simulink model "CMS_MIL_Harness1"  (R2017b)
settings: Solver=FixedStepDiscrete  StartTime=0.0  StopTime=23  FixedStep=0.01  RelTol=1e-3  EnableMultiTasking=on
undefined symbols (not defined in the file): sigbuilder_block
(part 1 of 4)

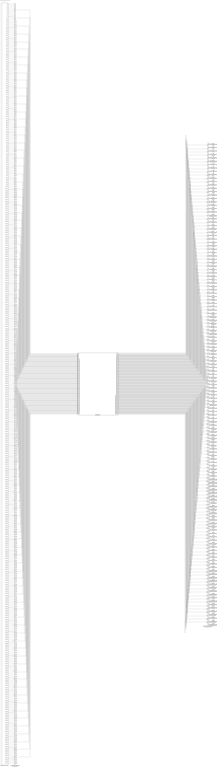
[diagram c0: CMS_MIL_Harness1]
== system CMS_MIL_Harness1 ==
  CMS_MIL : ModelReference  ModelNameDialog=CMS_MIL  SimulationMode=Normal  ModelReferenceVersion='M109C106'
  Harness Inputs : Subsystem  Tag=STV Subsys  LoadFcn=sigbuilder_block('load');  StartFcn=sigbuilder_block('start');  StopFcn=sigbuilder_block('stop');  ClipboardFcn=sigbuilder_block('clipboard');  mask(Sigbuilder block){tuvar=[0:10]}
      mask init:
      | if ~strcmp(get_param(bdroot(gcb),'SimulationStatus'),'stopped'),tuvar = sigbuilder_block('maskInit'); end
  Input Conversion Subsystem : Subsystem  Tag=__SLT_ICS__  Description=Signal spec. and routing
  Output Conversion Subsystem : Subsystem  Tag=__SLT_OCS__  Description=Signal spec. and routing
  GeCMS_HVConnSt_enum : Outport  OutDataTypeStr=uint8  PortDimensions=[1]
  GbCMS_NegCtlSt_flg : Outport  Port=2  OutDataTypeStr=boolean  PortDimensions=[1]
  GbCMS_PosCtlSt_flg : Outport  Port=3  OutDataTypeStr=boolean  PortDimensions=[1]
  GbCMS_ChrgPosCtlSt_flg : Outport  Port=4  OutDataTypeStr=boolean  PortDimensions=[1]
  GbCMS_ChrgNegCtlSt_flg : Outport  Port=5  OutDataTypeStr=boolean  PortDimensions=[1]
  GeCMS_RelStuckClosed_enum : Outport  Port=6  OutDataTypeStr=uint8  PortDimensions=[1]
  GcCMS_PackVolt_V : Outport  Port=7  OutDataTypeStr=fixdt('ufix16_Sp1')  PortDimensions=[1]
  GbCMS_PreChrgCtlSt_flg : Outport  Port=8  OutDataTypeStr=boolean  PortDimensions=[1]
  GcCMS_BattCurr_A : Outport  Port=9  OutDataTypeStr=fixdt('ufix16_Sp1_Bn700')  PortDimensions=[1]
  GbCMS_Kl15WkUp_flg : Outport  Port=10  OutDataTypeStr=boolean  PortDimensions=[1]
  GbCMS_ThmRunAway_flg : Outport  Port=11  OutDataTypeStr=boolean  PortDimensions=[1]
  GcCMS_CoolTempIn_C : Outport  Port=12  OutDataTypeStr=fixdt('ufix8_Bn40')  PortDimensions=[1]
  GcCMS_CoolTempOut_C : Outport  Port=13  OutDataTypeStr=fixdt('ufix8_Bn40')  PortDimensions=[1]
  GcCMS_CoolPwrReq_W : Outport  Port=14  OutDataTypeStr=fixdt('ufix16_Sp1')  PortDimensions=[1]
  GcCMS_HeatPwrReq_W : Outport  Port=15  OutDataTypeStr=fixdt('ufix16_Sp1')  PortDimensions=[1]
  GeCMS_CoolReq_enum : Outport  Port=16  OutDataTypeStr=uint8  PortDimensions=[1]
  GeCMS_HeatReq_enum : Outport  Port=17  OutDataTypeStr=uint8  PortDimensions=[1]
  GcCMS_PeakCurrDisCh_A : Outport  Port=18  OutDataTypeStr=fixdt('ufix16_Sp1')  PortDimensions=[1]
  GcCMS_PeakCurrCh_A : Outport  Port=19  OutDataTypeStr=fixdt('ufix16_Sp1_Bn1500')  PortDimensions=[1]
  GcCMS_PeakVoltDisCh_V : Outport  Port=20  OutDataTypeStr=uint16  PortDimensions=[1]
  GcCMS_PeakVoltCh_V : Outport  Port=21  OutDataTypeStr=uint16  PortDimensions=[1]
  GeCMS_Thm_propagat_enum : Outport  Port=22  OutDataTypeStr=uint8  PortDimensions=[1]
  GcCMS_ClntTgtTemp_C : Outport  Port=23  OutDataTypeStr=fixdt('ufix8_Bn40')  PortDimensions=[1]
  GcCMS_HtTgtTemp_C : Outport  Port=24  OutDataTypeStr=fixdt('ufix8_Bn40')  PortDimensions=[1]
  GcCMS_MaxCellVolt_V : Outport  Port=25  OutDataTypeStr=fixdt('ufix16_Sp001')  PortDimensions=[1]
  GcCMS_BusbarTempMax_C : Outport  Port=26  OutDataTypeStr=fixdt('ufix8_Bn40')  PortDimensions=[1]
  GcCMS_BusbarTempMin_C : Outport  Port=27  OutDataTypeStr=fixdt('ufix8_Bn40')  PortDimensions=[1]
  GcCMS_MinCellVolt_V : Outport  Port=28  OutDataTypeStr=fixdt('ufix16_Sp001')  PortDimensions=[1]
  GbCMS_ChrgCmd_flg : Outport  Port=29  OutDataTypeStr=boolean  PortDimensions=[1]
  GcCMS_ActPwrChrg_Kw : Outport  Port=30  OutDataTypeStr=fixdt('ufix16_Sp1')  PortDimensions=[1]
  GcCMS_MaxVoltChrg_V : Outport  Port=31  OutDataTypeStr=fixdt('ufix16_Sp1')  PortDimensions=[1]
  GcCMS_ReqVoltChrg_V : Outport  Port=32  OutDataTypeStr=fixdt('ufix16_Sp1')  PortDimensions=[1]
  GcCMS_ReqCurrChrg_A : Outport  Port=33  OutDataTypeStr=fixdt('ufix16_Sp1_Bn700')  PortDimensions=[1]
  GbCMS_ObcRdyReq_flg : Outport  Port=34  OutDataTypeStr=boolean  PortDimensions=[1]
  GbCMS_DischgCmd_flg : Outport  Port=35  OutDataTypeStr=boolean  PortDimensions=[1]
  GeCMS_BmsSt_enum : Outport  Port=36  OutDataTypeStr=uint8  PortDimensions=[1]
  GeCMS_BmsSelfChk_enum : Outport  Port=37  OutDataTypeStr=uint8  PortDimensions=[1]
  GeCMS_IsoFault_enum : Outport  Port=38  OutDataTypeStr=uint8  PortDimensions=[1]
  GcCMS_SocDspl_pct : Outport  Port=39  OutDataTypeStr=uint8  PortDimensions=[1]
  GbCMS_HvilOpenFault_flg : Outport  Port=40  OutDataTypeStr=boolean  PortDimensions=[1]
  GeCMS_FltLvl_enum : Outport  Port=41  OutDataTypeStr=uint8  PortDimensions=[1]
  GeCMS_V2xMod_enum : Outport  Port=42  OutDataTypeStr=uint8  PortDimensions=[1]
  GcCMS_ChgSOCset_pct : Outport  Port=43  OutDataTypeStr=fixdt('ufix8_B80')  PortDimensions=[1]
  GcCMS_BattSoh_pct : Outport  Port=44  OutDataTypeStr=uint8  PortDimensions=[1]
  GcCMS_SOCA_pct : Outport  Port=45  OutDataTypeStr=uint8  PortDimensions=[1]
  GeCMS_IviDischg_enum : Outport  Port=46  OutDataTypeStr=uint8  PortDimensions=[1]
  GcCMS_PackCurLem_A : Outport  Port=47  OutDataTypeStr=fixdt('ufix16_Bn1023')  PortDimensions=[1]
  GcCMS_BattInVolt_V : Outport  Port=48  OutDataTypeStr=fixdt('ufix16_Sp1')  PortDimensions=[1]
  GbCMS_BalSt_flg : Outport  Port=49  OutDataTypeStr=boolean  PortDimensions=[1]
  GbCMS_BalVlg_flg : Outport  Port=50  OutDataTypeStr=boolean  PortDimensions=[1]
  GbCMS_VcuPwrUpReq_flg : Outport  Port=51  OutDataTypeStr=boolean  PortDimensions=[1]
  GbCMS_VcuPwrUpReqVld_flg : Outport  Port=52  OutDataTypeStr=boolean  PortDimensions=[1]
  GcCMS_ConstCurrDisChMax_A : Outport  Port=53  OutDataTypeStr=fixdt('ufix16_Sp1')  PortDimensions=[1]
  GcCMS_ConstCurrChMax_A : Outport  Port=54  OutDataTypeStr=fixdt('ufix16_Sp1_Bn700')  PortDimensions=[1]
  GbCMS_PwrDownReq_flg : Outport  Port=55  OutDataTypeStr=boolean  PortDimensions=[1]
  GbCMS_PwrDownReqVld_flg : Outport  Port=56  OutDataTypeStr=boolean  PortDimensions=[1]
  GeCMS_ChrgPreThmMode_enum : Outport  Port=57  OutDataTypeStr=uint8  PortDimensions=[1]
  GeCMS_ElockReq_enum : Outport  Port=58  OutDataTypeStr=uint8  PortDimensions=[1]
  GeCMS_PreThmReq_enum : Outport  Port=59  OutDataTypeStr=uint8  PortDimensions=[1]
  GcCMS_PeakPwrDisCh_Kw : Outport  Port=60  OutDataTypeStr=fixdt('ufix16_Sp1')  PortDimensions=[1]
  GcCMS_PeakPwrCh_Kw : Outport  Port=61  OutDataTypeStr=fixdt('ufix16_Sp1')  PortDimensions=[1]
  GcCMS_ConstPwrDisCh_Kw : Outport  Port=62  OutDataTypeStr=fixdt('ufix16_Sp1')  PortDimensions=[1]
  GcCMS_ConstPwrCh_Kw : Outport  Port=63  OutDataTypeStr=fixdt('ufix16_Sp1')  PortDimensions=[1]
  GcCMS_ResIso_Kohm : Outport  Port=64  OutDataTypeStr=uint16  PortDimensions=[1]
  GcCMS_ChrgRemTime_Min : Outport  Port=65  OutDataTypeStr=uint16  PortDimensions=[1]
  GeCMS_ACPlugCnnt_enum : Outport  Port=66  OutDataTypeStr=uint8  PortDimensions=[1]
  GbCMS_BattFull_flg : Outport  Port=67  OutDataTypeStr=boolean  PortDimensions=[1]
  GbCMS_WarnLamp_flg : Outport  Port=68  OutDataTypeStr=boolean  PortDimensions=[1]
  GbCMS_SerLamp_flg : Outport  Port=69  OutDataTypeStr=boolean  PortDimensions=[1]
  GbCMS_TempDiffWarn_flg : Outport  Port=70  OutDataTypeStr=boolean  PortDimensions=[1]
  GbCMS_OverChrgWarn_flg : Outport  Port=71  OutDataTypeStr=boolean  PortDimensions=[1]
  GbCMS_ConsisWarn_flg : Outport  Port=72  OutDataTypeStr=boolean  PortDimensions=[1]
  GbCMS_MishWarn_flg : Outport  Port=73  OutDataTypeStr=boolean  PortDimensions=[1]
  GbCMS_SocHopWarn_flg : Outport  Port=74  OutDataTypeStr=boolean  PortDimensions=[1]
  GbCMS_SocHighWarn_flg : Outport  Port=75  OutDataTypeStr=boolean  PortDimensions=[1]
  GbCMS_SocLowWarn_flg : Outport  Port=76  OutDataTypeStr=boolean  PortDimensions=[1]
  GbCMS_OTAModeSt_flg : Outport  Port=77  OutDataTypeStr=boolean  PortDimensions=[1]
  GeCMS_AcDcConnBoth_enum : Outport  Port=78  OutDataTypeStr=uint8  PortDimensions=[1]
  GbCMS_CellUvFlt_flg : Outport  Port=79  OutDataTypeStr=boolean  PortDimensions=[1]
  GbCMS_CellOvFlt_flg : Outport  Port=80  OutDataTypeStr=boolean  PortDimensions=[1]
  GbCMS_PackUvFlt_flg : Outport  Port=81  OutDataTypeStr=boolean  PortDimensions=[1]
  GbCMS_PackOvFlt_flg : Outport  Port=82  OutDataTypeStr=boolean  PortDimensions=[1]
  GbCMS_TempHighWarn_flg : Outport  Port=83  OutDataTypeStr=boolean  PortDimensions=[1]
  GcCMS_RealSoc_pct : Outport  Port=84  OutDataTypeStr=uint8  PortDimensions=[1]
  GeCMS_DCPlugConn_enum : Outport  Port=85  OutDataTypeStr=uint8  PortDimensions=[1]
  GeCMS_ACChgMode_enum : Outport  Port=86  OutDataTypeStr=uint8  PortDimensions=[1]
  GeCMS_DCChgMode_enum : Outport  Port=87  OutDataTypeStr=uint8  PortDimensions=[1]
  GcCMS_BattTempAvrg_C : Outport  Port=88  OutDataTypeStr=fixdt('ufix8_Bn40')  PortDimensions=[1]
  GcCMS_BattNrmEnrg_kwh : Outport  Port=89  OutDataTypeStr=fixdt('ufix16_Sp01')  PortDimensions=[1]
  GbCMS_BattTempFault_flg : Outport  Port=90  OutDataTypeStr=boolean  PortDimensions=[1]
  GcCMS_BattSoe_kwh : Outport  Port=91  OutDataTypeStr=fixdt('ufix16_Sp1')  PortDimensions=[1]
  GbCMS_IsoChkSt_flg : Outport  Port=92  OutDataTypeStr=boolean  PortDimensions=[1]
  GcCMS_BattTempMax_C : Outport  Port=93  OutDataTypeStr=fixdt('ufix8_Bn40')  PortDimensions=[1]
  GcCMS_BattTempMin_C : Outport  Port=94  OutDataTypeStr=fixdt('ufix8_Bn40')  PortDimensions=[1]
  GcCMS_FuseVolt_V : Outport  Port=95  OutDataTypeStr=fixdt('ufix8_E1')  PortDimensions=[1]
  GcCMS_ChrgAccum_Ah : Outport  Port=96  OutDataTypeStr=uint8  PortDimensions=[1]
  GbCMS_DChgStVoltOut_flg : Outport  Port=97  OutDataTypeStr=boolean  PortDimensions=[1]
  GcCMS_DChrgVoltReq_V : Outport  Port=98  OutDataTypeStr=fixdt('ufix16_Sp1')  PortDimensions=[1]
  GcCMS_DChrgCurrReq_A : Outport  Port=99  OutDataTypeStr=fixdt('ufix16_Sp1_Bn400')  PortDimensions=[1]
  GcCMS_DChrgRchSocLmt_numb : Outport  Port=100  OutDataTypeStr=uint8  PortDimensions=[1]
  GcCMS_DChrgRchPackVoltLmt_numb : Outport  Port=101  OutDataTypeStr=uint8  PortDimensions=[1]
  GcCMS_DChrgRchCellVoltLmt_numb : Outport  Port=102  OutDataTypeStr=uint8  PortDimensions=[1]
  GcCMS_DChrgChrgerActStop_numb : Outport  Port=103  OutDataTypeStr=uint8  PortDimensions=[1]
  GcCMS_DChrgBattInsulationErr_numb : Outport  Port=104  OutDataTypeStr=uint8  PortDimensions=[1]
  GcCMS_DChrgOutpCnntOvrTempErr_numb : Outport  Port=105  OutDataTypeStr=uint8  PortDimensions=[1]
  GcCMS_PcbOvrTempErr_numb : Outport  Port=106  OutDataTypeStr=uint8  PortDimensions=[1]
  GcCMS_ChrgCnntErr_numb : Outport  Port=107  OutDataTypeStr=uint8  PortDimensions=[1]
  GcCMS_BattOvrTempErr_numb : Outport  Port=108  OutDataTypeStr=uint8  PortDimensions=[1]
  GcCMS_MainRelayErr_numb : Outport  Port=109  OutDataTypeStr=uint8  PortDimensions=[1]
  GcCMS_CC2ChkVoltErr_numb : Outport  Port=110  OutDataTypeStr=uint8  PortDimensions=[1]
  GcCMS_OtherErr_numb : Outport  Port=111  OutDataTypeStr=uint8  PortDimensions=[1]
  GcCMS_ChrgCurrAbnrm_numb : Outport  Port=112  OutDataTypeStr=uint8  PortDimensions=[1]
  GcCMS_ChrgVoltAbnrm_numb : Outport  Port=113  OutDataTypeStr=uint8  PortDimensions=[1]
  GcCMS_CellVoltCnt_numb : Outport  Port=114  OutDataTypeStr=uint8  PortDimensions=[1]
  GcCMS_CellVolt1_V : Outport  Port=115  OutDataTypeStr=fixdt('ufix16_Sp001')  PortDimensions=[1]
  GcCMS_CellVolt2_V : Outport  Port=116  OutDataTypeStr=fixdt('ufix16_Sp001')  PortDimensions=[1]
  GcCMS_CellVolt3_V : Outport  Port=117  OutDataTypeStr=fixdt('ufix16_Sp001')  PortDimensions=[1]
  GcCMS_CellVolt4_V : Outport  Port=118  OutDataTypeStr=fixdt('ufix16_Sp001')  PortDimensions=[1]
  GcCMS_CellTempCnt_numb : Outport  Port=119  OutDataTypeStr=uint8  PortDimensions=[1]
  GcCMS_CellTemp1_C : Outport  Port=120  OutDataTypeStr=fixdt('ufix8_Bn40')  PortDimensions=[1]
  GcCMS_CellTemp2_C : Outport  Port=121  OutDataTypeStr=fixdt('ufix8_Bn40')  PortDimensions=[1]
  GcCMS_CellTemp3_C : Outport  Port=122  OutDataTypeStr=fixdt('ufix8_Bn40')  PortDimensions=[1]
  GcCMS_CellTemp4_C : Outport  Port=123  OutDataTypeStr=fixdt('ufix8_Bn40')  PortDimensions=[1]
  GcCMS_CellTemp5_C : Outport  Port=124  OutDataTypeStr=fixdt('ufix8_Bn40')  PortDimensions=[1]
  GcCMS_CellTemp6_C : Outport  Port=125  OutDataTypeStr=fixdt('ufix8_Bn40')  PortDimensions=[1]
  GcCMS_CellTemp7_C : Outport  Port=126  OutDataTypeStr=fixdt('ufix8_Bn40')  PortDimensions=[1]
  GcCMS_MaxCellVoltNumb_numb : Outport  Port=127  OutDataTypeStr=uint8  PortDimensions=[1]
  GcCMS_MinCellVoltNumb_numb : Outport  Port=128  OutDataTypeStr=uint8  PortDimensions=[1]
  GcCMS_MaxCellTempNumb_numb : Outport  Port=129  OutDataTypeStr=uint8  PortDimensions=[1]
  GcCMS_MinCellTempNumb_numb : Outport  Port=130  OutDataTypeStr=uint8  PortDimensions=[1]
  GcCMS_MaxVoltNumb_numb : Outport  Port=131  OutDataTypeStr=uint8  PortDimensions=[1]
  GcCMS_MinVoltNumb_numb : Outport  Port=132  OutDataTypeStr=uint8  PortDimensions=[1]
  GcCMS_MaxTempNumb_numb : Outport  Port=133  OutDataTypeStr=uint8  PortDimensions=[1]
  GcCMS_MinTempNumb_numb : Outport  Port=134  OutDataTypeStr=uint8  PortDimensions=[1]
  GeCMS_ChgMode_enum : Outport  Port=135  OutDataTypeStr=uint8  PortDimensions=[1]
  GeCMS_DChrgModeDebug_enum : Outport  Port=136  OutDataTypeStr=uint8  PortDimensions=[1]
  GbCMS_DChrgWkUp_flg : Outport  Port=137  OutDataTypeStr=boolean  PortDimensions=[1]
  GeCMS_EvccMode_enum : Outport  Port=138  OutDataTypeStr=uint8  PortDimensions=[1]
  GeCMS_AChrgObsr_enum : Outport  Port=139  OutDataTypeStr=uint8  PortDimensions=[1]
  GeCMS_PreThmObsvr_enum : Outport  Port=140  OutDataTypeStr=uint8  PortDimensions=[1]
  GbCMS_StartCanSend_flg : Outport  Port=141  OutDataTypeStr=boolean  PortDimensions=[1]
  GeCMS_AppChgMode_enum : Outport  Port=142  OutDataTypeStr=uint8  PortDimensions=[1]
  GeCMS_DCchgIsolationFault_enum : Outport  Port=143  OutDataTypeStr=uint8  PortDimensions=[1]
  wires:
  Harness Inputs/1(GeCTC_CtrCtlState_enum) -> Input Conversion Subsystem/1(Inport_1)
  Harness Inputs/2(GbCTC_NegCtlState_flg) -> Input Conversion Subsystem/2(Inport_2)
  Harness Inputs/3(GbCTC_PosCtlState_flg) -> Input Conversion Subsystem/3(Inport_3)
  Harness Inputs/4(GbCTC_DCPosChrgCtlState_flg) -> Input Conversion Subsystem/4(Inport_4)
  Harness Inputs/5(GbCTC_DCNegChrgCtlState_flg) -> Input Conversion Subsystem/5(Inport_5)
  Harness Inputs/6(GcHDP_PackVolt_V) -> Input Conversion Subsystem/6(Inport_6)
  Harness Inputs/7(GbCTC_PreChrgCtlState_flg) -> Input Conversion Subsystem/7(Inport_7)
  Harness Inputs/8(GcHDP_PackCrnt_A) -> Input Conversion Subsystem/8(Inport_8)
  Harness Inputs/9(GbWSM_Kl15WkUpPrs_flg) -> Input Conversion Subsystem/9(Inport_9)
  Harness Inputs/10(GcCDP_MinCellVolt_mV) -> Input Conversion Subsystem/10(Inport_10)
  Harness Inputs/11(GcCDP_MaxCellVolt_mV) -> Input Conversion Subsystem/11(Inport_11)
  Harness Inputs/12(GbACC_ObcChrgCmd_flg) -> Input Conversion Subsystem/12(Inport_12)
  Harness Inputs/13(GcACC_ACChrgVoltRqst_V) -> Input Conversion Subsystem/13(Inport_13)
  Harness Inputs/14(GcACC_ACChrgCrntRqst_A) -> Input Conversion Subsystem/14(Inport_14)
  Harness Inputs/15(GbACC_ACChrgRqst_flg) -> Input Conversion Subsystem/15(Inport_15)
  Harness Inputs/16(GeCTC_CtrCtlConnMode_enum) -> Input Conversion Subsystem/16(Inport_16)
  Harness Inputs/17(GbMSM_SelfCheck_flg) -> Input Conversion Subsystem/17(Inport_17)
  Harness Inputs/18(GcSOC_DispSOC_pct) -> Input Conversion Subsystem/18(Inport_18)
  Harness Inputs/19(GbISP_TFHvilLFlt_flg) -> Input Conversion Subsystem/19(Inport_19)
  Harness Inputs/20(GeFTC_FltLvlOnCAN_enum) -> Input Conversion Subsystem/20(Inport_20)
  Harness Inputs/21(GcSOH_PackSOH_pct) -> Input Conversion Subsystem/21(Inport_21)
  Harness Inputs/22(GcSOC_PackSOC_pct) -> Input Conversion Subsystem/22(Inport_22)
  Harness Inputs/23(GcHDP_HallCrnt_A) -> Input Conversion Subsystem/23(Inport_23)
  Harness Inputs/24(GbMSM_SelfChckMaxTiReach_flg) -> Input Conversion Subsystem/24(Inport_24)
  Harness Inputs/25(GaCBC_CellBalCtlCmd_flg(1)) -> Input Conversion Subsystem/25(Inport_25)
  Harness Inputs/26(GaCBC_CellBalCtlCmd_flg(2)) -> Input Conversion Subsystem/26(Inport_26)
  Harness Inputs/27(GaCBC_CellBalCtlCmd_flg(3)) -> Input Conversion Subsystem/27(Inport_27)
  Harness Inputs/28(GaCBC_CellBalCtlCmd_flg(4)) -> Input Conversion Subsystem/28(Inport_28)
  Harness Inputs/29(GaCBC_CellBalCtlCmd_flg(5)) -> Input Conversion Subsystem/29(Inport_29)
  Harness Inputs/30(GaCBC_CellBalCtlCmd_flg(6)) -> Input Conversion Subsystem/30(Inport_30)
  Harness Inputs/31(GaCBC_CellBalCtlCmd_flg(7)) -> Input Conversion Subsystem/31(Inport_31)
  Harness Inputs/32(GaCBC_CellBalCtlCmd_flg(8)) -> Input Conversion Subsystem/32(Inport_32)
  Harness Inputs/33(GaCBC_CellBalCtlCmd_flg(9)) -> Input Conversion Subsystem/33(Inport_33)
  Harness Inputs/34(GaCBC_CellBalCtlCmd_flg(10)) -> Input Conversion Subsystem/34(Inport_34)
  Harness Inputs/35(GaCBC_CellBalCtlCmd_flg(11)) -> Input Conversion Subsystem/35(Inport_35)
  Harness Inputs/36(GaCBC_CellBalCtlCmd_flg(12)) -> Input Conversion Subsystem/36(Inport_36)
  Harness Inputs/37(GaCBC_CellBalCtlCmd_flg(13)) -> Input Conversion Subsystem/37(Inport_37)
  Harness Inputs/38(GaCBC_CellBalCtlCmd_flg(14)) -> Input Conversion Subsystem/38(Inport_38)
  Harness Inputs/39(GaCBC_CellBalCtlCmd_flg(15)) -> Input Conversion Subsystem/39(Inport_39)
  Harness Inputs/40(GaCBC_CellBalCtlCmd_flg(16)) -> Input Conversion Subsystem/40(Inport_40)
  Harness Inputs/41(GaCBC_CellBalCtlCmd_flg(17)) -> Input Conversion Subsystem/41(Inport_41)
  Harness Inputs/42(GaCBC_CellBalCtlCmd_flg(18)) -> Input Conversion Subsystem/42(Inport_42)
  Harness Inputs/43(GaCBC_CellBalCtlCmd_flg(19)) -> Input Conversion Subsystem/43(Inport_43)
  Harness Inputs/44(GaCBC_CellBalCtlCmd_flg(20)) -> Input Conversion Subsystem/44(Inport_44)
  Harness Inputs/45(GaCBC_CellBalCtlCmd_flg(21)) -> Input Conversion Subsystem/45(Inport_45)
  Harness Inputs/46(GaCBC_CellBalCtlCmd_flg(22)) -> Input Conversion Subsystem/46(Inport_46)
  Harness Inputs/47(GaCBC_CellBalCtlCmd_flg(23)) -> Input Conversion Subsystem/47(Inport_47)
  Harness Inputs/48(GaCBC_CellBalCtlCmd_flg(24)) -> Input Conversion Subsystem/48(Inport_48)
  Harness Inputs/49(GaCBC_CellBalCtlCmd_flg(25)) -> Input Conversion Subsystem/49(Inport_49)
  Harness Inputs/50(GaCBC_CellBalCtlCmd_flg(26)) -> Input Conversion Subsystem/50(Inport_50)
  Harness Inputs/51(GaCBC_CellBalCtlCmd_flg(27)) -> Input Conversion Subsystem/51(Inport_51)
  Harness Inputs/52(GaCBC_CellBalCtlCmd_flg(28)) -> Input Conversion Subsystem/52(Inport_52)
  Harness Inputs/53(GaCBC_CellBalCtlCmd_flg(29)) -> Input Conversion Subsystem/53(Inport_53)
  Harness Inputs/54(GaCBC_CellBalCtlCmd_flg(30)) -> Input Conversion Subsystem/54(Inport_54)
  Harness Inputs/55(GaCBC_CellBalCtlCmd_flg(31)) -> Input Conversion Subsystem/55(Inport_55)
  Harness Inputs/56(GaCBC_CellBalCtlCmd_flg(32)) -> Input Conversion Subsystem/56(Inport_56)
  Harness Inputs/57(GaCBC_CellBalCtlCmd_flg(33)) -> Input Conversion Subsystem/57(Inport_57)
  Harness Inputs/58(GaCBC_CellBalCtlCmd_flg(34)) -> Input Conversion Subsystem/58(Inport_58)
  Harness Inputs/59(GaCBC_CellBalCtlCmd_flg(35)) -> Input Conversion Subsystem/59(Inport_59)
  Harness Inputs/60(GaCBC_CellBalCtlCmd_flg(36)) -> Input Conversion Subsystem/60(Inport_60)
  Harness Inputs/61(GaCBC_CellBalCtlCmd_flg(37)) -> Input Conversion Subsystem/61(Inport_61)
  Harness Inputs/62(GaCBC_CellBalCtlCmd_flg(38)) -> Input Conversion Subsystem/62(Inport_62)
  Harness Inputs/63(GaCBC_CellBalCtlCmd_flg(39)) -> Input Conversion Subsystem/63(Inport_63)
  Harness Inputs/64(GaCBC_CellBalCtlCmd_flg(40)) -> Input Conversion Subsystem/64(Inport_64)
  Harness Inputs/65(GaCBC_CellBalCtlCmd_flg(41)) -> Input Conversion Subsystem/65(Inport_65)
  Harness Inputs/66(GaCBC_CellBalCtlCmd_flg(42)) -> Input Conversion Subsystem/66(Inport_66)
  Harness Inputs/67(GaCBC_CellBalCtlCmd_flg(43)) -> Input Conversion Subsystem/67(Inport_67)
  Harness Inputs/68(GaCBC_CellBalCtlCmd_flg(44)) -> Input Conversion Subsystem/68(Inport_68)
  Harness Inputs/69(GaCBC_CellBalCtlCmd_flg(45)) -> Input Conversion Subsystem/69(Inport_69)
  Harness Inputs/70(GaCBC_CellBalCtlCmd_flg(46)) -> Input Conversion Subsystem/70(Inport_70)
  Harness Inputs/71(GaCBC_CellBalCtlCmd_flg(47)) -> Input Conversion Subsystem/71(Inport_71)
  Harness Inputs/72(GaCBC_CellBalCtlCmd_flg(48)) -> Input Conversion Subsystem/72(Inport_72)
  Harness Inputs/73(GaCBC_CellBalCtlCmd_flg(49)) -> Input Conversion Subsystem/73(Inport_73)
  Harness Inputs/74(GaCBC_CellBalCtlCmd_flg(50)) -> Input Conversion Subsystem/74(Inport_74)
  Harness Inputs/75(GaCBC_CellBalCtlCmd_flg(51)) -> Input Conversion Subsystem/75(Inport_75)
  Harness Inputs/76(GaCBC_CellBalCtlCmd_flg(52)) -> Input Conversion Subsystem/76(Inport_76)
  Harness Inputs/77(GaCBC_CellBalCtlCmd_flg(53)) -> Input Conversion Subsystem/77(Inport_77)
  Harness Inputs/78(GaCBC_CellBalCtlCmd_flg(54)) -> Input Conversion Subsystem/78(Inport_78)
  Harness Inputs/79(GaCBC_CellBalCtlCmd_flg(55)) -> Input Conversion Subsystem/79(Inport_79)
  Harness Inputs/80(GaCBC_CellBalCtlCmd_flg(56)) -> Input Conversion Subsystem/80(Inport_80)
  Harness Inputs/81(GaCBC_CellBalCtlCmd_flg(57)) -> Input Conversion Subsystem/81(Inport_81)
  Harness Inputs/82(GaCBC_CellBalCtlCmd_flg(58)) -> Input Conversion Subsystem/82(Inport_82)
  Harness Inputs/83(GaCBC_CellBalCtlCmd_flg(59)) -> Input Conversion Subsystem/83(Inport_83)
  Harness Inputs/84(GaCBC_CellBalCtlCmd_flg(60)) -> Input Conversion Subsystem/84(Inport_84)
  Harness Inputs/85(GaCBC_CellBalCtlCmd_flg(61)) -> Input Conversion Subsystem/85(Inport_85)
  Harness Inputs/86(GaCBC_CellBalCtlCmd_flg(62)) -> Input Conversion Subsystem/86(Inport_86)
  Harness Inputs/87(GaCBC_CellBalCtlCmd_flg(63)) -> Input Conversion Subsystem/87(Inport_87)
  Harness Inputs/88(GaCBC_CellBalCtlCmd_flg(64)) -> Input Conversion Subsystem/88(Inport_88)
  Harness Inputs/89(GaCBC_CellBalCtlCmd_flg(65)) -> Input Conversion Subsystem/89(Inport_89)
  Harness Inputs/90(GaCBC_CellBalCtlCmd_flg(66)) -> Input Conversion Subsystem/90(Inport_90)
  Harness Inputs/91(GaCBC_CellBalCtlCmd_flg(67)) -> Input Conversion Subsystem/91(Inport_91)
  Harness Inputs/92(GaCBC_CellBalCtlCmd_flg(68)) -> Input Conversion Subsystem/92(Inport_92)
  Harness Inputs/93(GaCBC_CellBalCtlCmd_flg(69)) -> Input Conversion Subsystem/93(Inport_93)
  Harness Inputs/94(GaCBC_CellBalCtlCmd_flg(70)) -> Input Conversion Subsystem/94(Inport_94)
  Harness Inputs/95(GaCBC_CellBalCtlCmd_flg(71)) -> Input Conversion Subsystem/95(Inport_95)
  Harness Inputs/96(GaCBC_CellBalCtlCmd_flg(72)) -> Input Conversion Subsystem/96(Inport_96)
  Harness Inputs/97(GaCBC_CellBalCtlCmd_flg(73)) -> Input Conversion Subsystem/97(Inport_97)
  Harness Inputs/98(GaCBC_CellBalCtlCmd_flg(74)) -> Input Conversion Subsystem/98(Inport_98)
  Harness Inputs/99(GaCBC_CellBalCtlCmd_flg(75)) -> Input Conversion Subsystem/99(Inport_99)
  Harness Inputs/100(GaCBC_CellBalCtlCmd_flg(76)) -> Input Conversion Subsystem/100(Inport_100)
  Harness Inputs/101(GaCBC_CellBalCtlCmd_flg(77)) -> Input Conversion Subsystem/101(Inport_101)
  Harness Inputs/102(GaCBC_CellBalCtlCmd_flg(78)) -> Input Conversion Subsystem/102(Inport_102)
  Harness Inputs/103(GaCBC_CellBalCtlCmd_flg(79)) -> Input Conversion Subsystem/103(Inport_103)
  Harness Inputs/104(GaCBC_CellBalCtlCmd_flg(80)) -> Input Conversion Subsystem/104(Inport_104)
  Harness Inputs/105(GaCBC_CellBalCtlCmd_flg(81)) -> Input Conversion Subsystem/105(Inport_105)
  Harness Inputs/106(GaCBC_CellBalCtlCmd_flg(82)) -> Input Conversion Subsystem/106(Inport_106)
  Harness Inputs/107(GaCBC_CellBalCtlCmd_flg(83)) -> Input Conversion Subsystem/107(Inport_107)
  Harness Inputs/108(GaCBC_CellBalCtlCmd_flg(84)) -> Input Conversion Subsystem/108(Inport_108)
  Harness Inputs/109(GaCBC_CellBalCtlCmd_flg(85)) -> Input Conversion Subsystem/109(Inport_109)
  Harness Inputs/110(GaCBC_CellBalCtlCmd_flg(86)) -> Input Conversion Subsystem/110(Inport_110)
  Harness Inputs/111(GaCBC_CellBalCtlCmd_flg(87)) -> Input Conversion Subsystem/111(Inport_111)
  Harness Inputs/112(GaCBC_CellBalCtlCmd_flg(88)) -> Input Conversion Subsystem/112(Inport_112)
  Harness Inputs/113(GaCBC_CellBalCtlCmd_flg(89)) -> Input Conversion Subsystem/113(Inport_113)
  Harness Inputs/114(GaCBC_CellBalCtlCmd_flg(90)) -> Input Conversion Subsystem/114(Inport_114)
  Harness Inputs/115(GaCBC_CellBalCtlCmd_flg(91)) -> Input Conversion Subsystem/115(Inport_115)
  Harness Inputs/116(GaCBC_CellBalCtlCmd_flg(92)) -> Input Conversion Subsystem/116(Inport_116)
  Harness Inputs/117(GaCBC_CellBalCtlCmd_flg(93)) -> Input Conversion Subsystem/117(Inport_117)
  Harness Inputs/118(GaCBC_CellBalCtlCmd_flg(94)) -> Input Conversion Subsystem/118(Inport_118)
  Harness Inputs/119(GaCBC_CellBalCtlCmd_flg(95)) -> Input Conversion Subsystem/119(Inport_119)
  Harness Inputs/120(GaCBC_CellBalCtlCmd_flg(96)) -> Input Conversion Subsystem/120(Inport_120)
  Harness Inputs/121(GaCBC_CellBalCtlCmd_flg(97)) -> Input Conversion Subsystem/121(Inport_121)
  Harness Inputs/122(GaCBC_CellBalCtlCmd_flg(98)) -> Input Conversion Subsystem/122(Inport_122)
  Harness Inputs/123(GaCBC_CellBalCtlCmd_flg(99)) -> Input Conversion Subsystem/123(Inport_123)
  Harness Inputs/124(GaCBC_CellBalCtlCmd_flg(100)) -> Input Conversion Subsystem/124(Inport_124)
  Harness Inputs/125(GaCBC_CellBalCtlCmd_flg(101)) -> Input Conversion Subsystem/125(Inport_125)
  Harness Inputs/126(GaCBC_CellBalCtlCmd_flg(102)) -> Input Conversion Subsystem/126(Inport_126)
  Harness Inputs/127(GaCBC_CellBalCtlCmd_flg(103)) -> Input Conversion Subsystem/127(Inport_127)
  Harness Inputs/128(GaCBC_CellBalCtlCmd_flg(104)) -> Input Conversion Subsystem/128(Inport_128)
  Harness Inputs/129(GaCBC_CellBalCtlCmd_flg(105)) -> Input Conversion Subsystem/129(Inport_129)
  Harness Inputs/130(GaCBC_CellBalCtlCmd_flg(106)) -> Input Conversion Subsystem/130(Inport_130)
  Harness Inputs/131(GaCBC_CellBalCtlCmd_flg(107)) -> Input Conversion Subsystem/131(Inport_131)
  Harness Inputs/132(GaCBC_CellBalCtlCmd_flg(108)) -> Input Conversion Subsystem/132(Inport_132)
  Harness Inputs/133(GaCBC_CellBalCtlCmd_flg(109)) -> Input Conversion Subsystem/133(Inport_133)
  Harness Inputs/134(GaCBC_CellBalCtlCmd_flg(110)) -> Input Conversion Subsystem/134(Inport_134)
  Harness Inputs/135(GaCBC_CellBalCtlCmd_flg(111)) -> Input Conversion Subsystem/135(Inport_135)
  Harness Inputs/136(GaCBC_CellBalCtlCmd_flg(112)) -> Input Conversion Subsystem/136(Inport_136)
  Harness Inputs/137(GbDCC_DCChrgRqst_flg) -> Input Conversion Subsystem/137(Inport_137)
  Harness Inputs/138(GcSOP_DischrgConstPwr_kW) -> Input Conversion Subsystem/138(Inport_138)
  Harness Inputs/139(GcSOP_ChrgConstPwr_kW) -> Input Conversion Subsystem/139(Inport_139)
  Harness Inputs/140(GcISO_HVIsoValue_kohm) -> Input Conversion Subsystem/140(Inport_140)
  Harness Inputs/141(GeODP_ObcCcSt_enum) -> Input Conversion Subsystem/141(Inport_141)
  Harness Inputs/142(GbDCC_DCChrgFinish_flg) -> Input Conversion Subsystem/142(Inport_142)
  Harness Inputs/143(GbACC_ACChrgFinish_flg) -> Input Conversion Subsystem/143(Inport_143)
  Harness Inputs/144(GeACC_ACChrgState_enum) -> Input Conversion Subsystem/144(Inport_144)
  Harness Inputs/145(GeDCC_DCConnSt_enum) -> Input Conversion Subsystem/145(Inport_145)
  Harness Inputs/146(GeLDP_CC2St_enum) -> Input Conversion Subsystem/146(Inport_146)
  Harness Inputs/147(GcCDP_AvgCellTemp_C) -> Input Conversion Subsystem/147(Inport_147)
  Harness Inputs/148(GbISO_IsoForbid_flg) -> Input Conversion Subsystem/148(Inport_148)
  Harness Inputs/149(GcCDP_MaxCellTemp_C) -> Input Conversion Subsystem/149(Inport_149)
  Harness Inputs/150(GcCDP_MinCellTemp_C) -> Input Conversion Subsystem/150(Inport_150)
  Harness Inputs/151(GcDCS_3072ChrgVoltReq_V) -> Input Conversion Subsystem/151(Inport_151)
  Harness Inputs/152(GcDCC_DCChrgCrntRqst_A) -> Input Conversion Subsystem/152(Inport_152)
  Harness Inputs/153(GaCDP_CellVolt_mV(1)) -> Input Conversion Subsystem/153(Inport_153)
  Harness Inputs/154(GaCDP_CellVolt_mV(2)) -> Input Conversion Subsystem/154(Inport_154)
  Harness Inputs/155(GaCDP_CellVolt_mV(3)) -> Input Conversion Subsystem/155(Inport_155)
  Harness Inputs/156(GaCDP_CellVolt_mV(4)) -> Input Conversion Subsystem/156(Inport_156)
  Harness Inputs/157(GaCDP_CellVolt_mV(5)) -> Input Conversion Subsystem/157(Inport_157)
  Harness Inputs/158(GaCDP_CellVolt_mV(6)) -> Input Conversion Subsystem/158(Inport_158)
  Harness Inputs/159(GaCDP_CellVolt_mV(7)) -> Input Conversion Subsystem/159(Inport_159)
  Harness Inputs/160(GaCDP_CellVolt_mV(8)) -> Input Conversion Subsystem/160(Inport_160)
  Harness Inputs/161(GaCDP_CellVolt_mV(9)) -> Input Conversion Subsystem/161(Inport_161)
  Harness Inputs/162(GaCDP_CellVolt_mV(10)) -> Input Conversion Subsystem/162(Inport_162)
  Harness Inputs/163(GaCDP_CellVolt_mV(11)) -> Input Conversion Subsystem/163(Inport_163)
  Harness Inputs/164(GaCDP_CellVolt_mV(12)) -> Input Conversion Subsystem/164(Inport_164)
  Harness Inputs/165(GaCDP_CellVolt_mV(13)) -> Input Conversion Subsystem/165(Inport_165)
  Harness Inputs/166(GaCDP_CellVolt_mV(14)) -> Input Conversion Subsystem/166(Inport_166)
  Harness Inputs/167(GaCDP_CellVolt_mV(15)) -> Input Conversion Subsystem/167(Inport_167)
  Harness Inputs/168(GaCDP_CellVolt_mV(16)) -> Input Conversion Subsystem/168(Inport_168)
  Harness Inputs/169(GaCDP_CellVolt_mV(17)) -> Input Conversion Subsystem/169(Inport_169)
  Harness Inputs/170(GaCDP_CellVolt_mV(18)) -> Input Conversion Subsystem/170(Inport_170)
  Harness Inputs/171(GaCDP_CellVolt_mV(19)) -> Input Conversion Subsystem/171(Inport_171)
  Harness Inputs/172(GaCDP_CellVolt_mV(20)) -> Input Conversion Subsystem/172(Inport_172)
  Harness Inputs/173(GaCDP_CellVolt_mV(21)) -> Input Conversion Subsystem/173(Inport_173)
  Harness Inputs/174(GaCDP_CellVolt_mV(22)) -> Input Conversion Subsystem/174(Inport_174)
  Harness Inputs/175(GaCDP_CellVolt_mV(23)) -> Input Conversion Subsystem/175(Inport_175)
  Harness Inputs/176(GaCDP_CellVolt_mV(24)) -> Input Conversion Subsystem/176(Inport_176)
  Harness Inputs/177(GaCDP_CellVolt_mV(25)) -> Input Conversion Subsystem/177(Inport_177)
  Harness Inputs/178(GaCDP_CellVolt_mV(26)) -> Input Conversion Subsystem/178(Inport_178)
  Harness Inputs/179(GaCDP_CellVolt_mV(27)) -> Input Conversion Subsystem/179(Inport_179)
  Harness Inputs/180(GaCDP_CellVolt_mV(28)) -> Input Conversion Subsystem/180(Inport_180)
  Harness Inputs/181(GaCDP_CellVolt_mV(29)) -> Input Conversion Subsystem/181(Inport_181)
  Harness Inputs/182(GaCDP_CellVolt_mV(30)) -> Input Conversion Subsystem/182(Inport_182)
  Harness Inputs/183(GaCDP_CellVolt_mV(31)) -> Input Conversion Subsystem/183(Inport_183)
  Harness Inputs/184(GaCDP_CellVolt_mV(32)) -> Input Conversion Subsystem/184(Inport_184)
  Harness Inputs/185(GaCDP_CellVolt_mV(33)) -> Input Conversion Subsystem/185(Inport_185)
  Harness Inputs/186(GaCDP_CellVolt_mV(34)) -> Input Conversion Subsystem/186(Inport_186)
  Harness Inputs/187(GaCDP_CellVolt_mV(35)) -> Input Conversion Subsystem/187(Inport_187)
  Harness Inputs/188(GaCDP_CellVolt_mV(36)) -> Input Conversion Subsystem/188(Inport_188)
  Harness Inputs/189(GaCDP_CellVolt_mV(37)) -> Input Conversion Subsystem/189(Inport_189)
  Harness Inputs/190(GaCDP_CellVolt_mV(38)) -> Input Conversion Subsystem/190(Inport_190)
  Harness Inputs/191(GaCDP_CellVolt_mV(39)) -> Input Conversion Subsystem/191(Inport_191)
  Harness Inputs/192(GaCDP_CellVolt_mV(40)) -> Input Conversion Subsystem/192(Inport_192)
  Harness Inputs/193(GaCDP_CellVolt_mV(41)) -> Input Conversion Subsystem/193(Inport_193)
  Harness Inputs/194(GaCDP_CellVolt_mV(42)) -> Input Conversion Subsystem/194(Inport_194)
  Harness Inputs/195(GaCDP_CellVolt_mV(43)) -> Input Conversion Subsystem/195(Inport_195)
  Harness Inputs/196(GaCDP_CellVolt_mV(44)) -> Input Conversion Subsystem/196(Inport_196)
  Harness Inputs/197(GaCDP_CellVolt_mV(45)) -> Input Conversion Subsystem/197(Inport_197)
  Harness Inputs/198(GaCDP_CellVolt_mV(46)) -> Input Conversion Subsystem/198(Inport_198)
  Harness Inputs/199(GaCDP_CellVolt_mV(47)) -> Input Conversion Subsystem/199(Inport_199)
  Harness Inputs/200(GaCDP_CellVolt_mV(48)) -> Input Conversion Subsystem/200(Inport_200)
  Harness Inputs/201(GaCDP_CellVolt_mV(49)) -> Input Conversion Subsystem/201(Inport_201)
  Harness Inputs/202(GaCDP_CellVolt_mV(50)) -> Input Conversion Subsystem/202(Inport_202)
  Harness Inputs/203(GaCDP_CellVolt_mV(51)) -> Input Conversion Subsystem/203(Inport_203)
  Harness Inputs/204(GaCDP_CellVolt_mV(52)) -> Input Conversion Subsystem/204(Inport_204)
  Harness Inputs/205(GaCDP_CellVolt_mV(53)) -> Input Conversion Subsystem/205(Inport_205)
  Harness Inputs/206(GaCDP_CellVolt_mV(54)) -> Input Conversion Subsystem/206(Inport_206)
  Harness Inputs/207(GaCDP_CellVolt_mV(55)) -> Input Conversion Subsystem/207(Inport_207)
  Harness Inputs/208(GaCDP_CellVolt_mV(56)) -> Input Conversion Subsystem/208(Inport_208)
  Harness Inputs/209(GaCDP_CellVolt_mV(57)) -> Input Conversion Subsystem/209(Inport_209)
  Harness Inputs/210(GaCDP_CellVolt_mV(58)) -> Input Conversion Subsystem/210(Inport_210)
  Harness Inputs/211(GaCDP_CellVolt_mV(59)) -> Input Conversion Subsystem/211(Inport_211)
  Harness Inputs/212(GaCDP_CellVolt_mV(60)) -> Input Conversion Subsystem/212(Inport_212)
  Harness Inputs/213(GaCDP_CellVolt_mV(61)) -> Input Conversion Subsystem/213(Inport_213)
  Harness Inputs/214(GaCDP_CellVolt_mV(62)) -> Input Conversion Subsystem/214(Inport_214)
  Harness Inputs/215(GaCDP_CellVolt_mV(63)) -> Input Conversion Subsystem/215(Inport_215)
  Harness Inputs/216(GaCDP_CellVolt_mV(64)) -> Input Conversion Subsystem/216(Inport_216)
  Harness Inputs/217(GaCDP_CellVolt_mV(65)) -> Input Conversion Subsystem/217(Inport_217)
  Harness Inputs/218(GaCDP_CellVolt_mV(66)) -> Input Conversion Subsystem/218(Inport_218)
  Harness Inputs/219(GaCDP_CellVolt_mV(67)) -> Input Conversion Subsystem/219(Inport_219)
  Harness Inputs/220(GaCDP_CellVolt_mV(68)) -> Input Conversion Subsystem/220(Inport_220)
  Harness Inputs/221(GaCDP_CellVolt_mV(69)) -> Input Conversion Subsystem/221(Inport_221)
  Harness Inputs/222(GaCDP_CellVolt_mV(70)) -> Input Conversion Subsystem/222(Inport_222)
  Harness Inputs/223(GaCDP_CellVolt_mV(71)) -> Input Conversion Subsystem/223(Inport_223)
  Harness Inputs/224(GaCDP_CellVolt_mV(72)) -> Input Conversion Subsystem/224(Inport_224)
  Harness Inputs/225(GaCDP_CellVolt_mV(73)) -> Input Conversion Subsystem/225(Inport_225)
  Harness Inputs/226(GaCDP_CellVolt_mV(74)) -> Input Conversion Subsystem/226(Inport_226)
  Harness Inputs/227(GaCDP_CellVolt_mV(75)) -> Input Conversion Subsystem/227(Inport_227)
  Harness Inputs/228(GaCDP_CellVolt_mV(76)) -> Input Conversion Subsystem/228(Inport_228)
  Harness Inputs/229(GaCDP_CellVolt_mV(77)) -> Input Conversion Subsystem/229(Inport_229)
  Harness Inputs/230(GaCDP_CellVolt_mV(78)) -> Input Conversion Subsystem/230(Inport_230)
  Harness Inputs/231(GaCDP_CellVolt_mV(79)) -> Input Conversion Subsystem/231(Inport_231)
  Harness Inputs/232(GaCDP_CellVolt_mV(80)) -> Input Conversion Subsystem/232(Inport_232)
  Harness Inputs/233(GaCDP_CellVolt_mV(81)) -> Input Conversion Subsystem/233(Inport_233)
  Harness Inputs/234(GaCDP_CellVolt_mV(82)) -> Input Conversion Subsystem/234(Inport_234)
  Harness Inputs/235(GaCDP_CellVolt_mV(83)) -> Input Conversion Subsystem/235(Inport_235)
  Harness Inputs/236(GaCDP_CellVolt_mV(84)) -> Input Conversion Subsystem/236(Inport_236)
  Harness Inputs/237(GaCDP_CellVolt_mV(85)) -> Input Conversion Subsystem/237(Inport_237)
  Harness Inputs/238(GaCDP_CellVolt_mV(86)) -> Input Conversion Subsystem/238(Inport_238)
  Harness Inputs/239(GaCDP_CellVolt_mV(87)) -> Input Conversion Subsystem/239(Inport_239)
  Harness Inputs/240(GaCDP_CellVolt_mV(88)) -> Input Conversion Subsystem/240(Inport_240)
  Harness Inputs/241(GaCDP_CellVolt_mV(89)) -> Input Conversion Subsystem/241(Inport_241)
  Harness Inputs/242(GaCDP_CellVolt_mV(90)) -> Input Conversion Subsystem/242(Inport_242)
  Harness Inputs/243(GaCDP_CellVolt_mV(91)) -> Input Conversion Subsystem/243(Inport_243)
  Harness Inputs/244(GaCDP_CellVolt_mV(92)) -> Input Conversion Subsystem/244(Inport_244)
  Harness Inputs/245(GaCDP_CellVolt_mV(93)) -> Input Conversion Subsystem/245(Inport_245)
  Harness Inputs/246(GaCDP_CellVolt_mV(94)) -> Input Conversion Subsystem/246(Inport_246)
  Harness Inputs/247(GaCDP_CellVolt_mV(95)) -> Input Conversion Subsystem/247(Inport_247)
  Harness Inputs/248(GaCDP_CellVolt_mV(96)) -> Input Conversion Subsystem/248(Inport_248)
  Harness Inputs/249(GaCDP_CellVolt_mV(97)) -> Input Conversion Subsystem/249(Inport_249)
  Harness Inputs/250(GaCDP_CellVolt_mV(98)) -> Input Conversion Subsystem/250(Inport_250)
  Harness Inputs/251(GaCDP_CellVolt_mV(99)) -> Input Conversion Subsystem/251(Inport_251)
  Harness Inputs/252(GaCDP_CellVolt_mV(100)) -> Input Conversion Subsystem/252(Inport_252)
  Harness Inputs/253(GaCDP_CellVolt_mV(101)) -> Input Conversion Subsystem/253(Inport_253)
  Harness Inputs/254(GaCDP_CellVolt_mV(102)) -> Input Conversion Subsystem/254(Inport_254)
  Harness Inputs/255(GaCDP_CellVolt_mV(103)) -> Input Conversion Subsystem/255(Inport_255)
  Harness Inputs/256(GaCDP_CellVolt_mV(104)) -> Input Conversion Subsystem/256(Inport_256)
  Harness Inputs/257(GaCDP_CellVolt_mV(105)) -> Input Conversion Subsystem/257(Inport_257)
  Harness Inputs/258(GaCDP_CellVolt_mV(106)) -> Input Conversion Subsystem/258(Inport_258)
  Harness Inputs/259(GaCDP_CellVolt_mV(107)) -> Input Conversion Subsystem/259(Inport_259)
  Harness Inputs/260(GaCDP_CellVolt_mV(108)) -> Input Conversion Subsystem/260(Inport_260)
  Harness Inputs/261(GaCDP_CellVolt_mV(109)) -> Input Conversion Subsystem/261(Inport_261)
  Harness Inputs/262(GaCDP_CellVolt_mV(110)) -> Input Conversion Subsystem/262(Inport_262)
  Harness Inputs/263(GaCDP_CellVolt_mV(111)) -> Input Conversion Subsystem/263(Inport_263)
  Harness Inputs/264(GaCDP_CellVolt_mV(112)) -> Input Conversion Subsystem/264(Inport_264)
  Harness Inputs/265(GaCDP_CellTemp_C(1)) -> Input Conversion Subsystem/265(Inport_265)
  Harness Inputs/266(GaCDP_CellTemp_C(2)) -> Input Conversion Subsystem/266(Inport_266)
  Harness Inputs/267(GaCDP_CellTemp_C(3)) -> Input Conversion Subsystem/267(Inport_267)
  Harness Inputs/268(GaCDP_CellTemp_C(4)) -> Input Conversion Subsystem/268(Inport_268)
  Harness Inputs/269(GaCDP_CellTemp_C(5)) -> Input Conversion Subsystem/269(Inport_269)
  Harness Inputs/270(GaCDP_CellTemp_C(6)) -> Input Conversion Subsystem/270(Inport_270)
  Harness Inputs/271(GaCDP_CellTemp_C(7)) -> Input Conversion Subsystem/271(Inport_271)
  Harness Inputs/272(GaCDP_CellTemp_C(8)) -> Input Conversion Subsystem/272(Inport_272)
  Harness Inputs/273(GaCDP_CellTemp_C(9)) -> Input Conversion Subsystem/273(Inport_273)
  Harness Inputs/274(GaCDP_CellTemp_C(10)) -> Input Conversion Subsystem/274(Inport_274)
  Harness Inputs/275(GaCDP_CellTemp_C(11)) -> Input Conversion Subsystem/275(Inport_275)
  Harness Inputs/276(GaCDP_CellTemp_C(12)) -> Input Conversion Subsystem/276(Inport_276)
  Harness Inputs/277(GaCDP_CellTemp_C(13)) -> Input Conversion Subsystem/277(Inport_277)
  Harness Inputs/278(GaCDP_CellTemp_C(14)) -> Input Conversion Subsystem/278(Inport_278)
  Harness Inputs/279(GaCDP_CellTemp_C(15)) -> Input Conversion Subsystem/279(Inport_279)
  Harness Inputs/280(GaCDP_CellTemp_C(16)) -> Input Conversion Subsystem/280(Inport_280)
  Harness Inputs/281(GaCDP_CellTemp_C(17)) -> Input Conversion Subsystem/281(Inport_281)
  Harness Inputs/282(GaCDP_CellTemp_C(18)) -> Input Conversion Subsystem/282(Inport_282)
  Harness Inputs/283(GaCDP_CellTemp_C(19)) -> Input Conversion Subsystem/283(Inport_283)
  Harness Inputs/284(GaCDP_CellTemp_C(20)) -> Input Conversion Subsystem/284(Inport_284)
  Harness Inputs/285(GaCDP_CellTemp_C(21)) -> Input Conversion Subsystem/285(Inport_285)
  Harness Inputs/286(GaCDP_CellTemp_C(22)) -> Input Conversion Subsystem/286(Inport_286)
  Harness Inputs/287(GaCDP_CellTemp_C(23)) -> Input Conversion Subsystem/287(Inport_287)
  Harness Inputs/288(GaCDP_CellTemp_C(24)) -> Input Conversion Subsystem/288(Inport_288)
  Harness Inputs/289(GaCDP_CellTemp_C(25)) -> Input Conversion Subsystem/289(Inport_289)
  Harness Inputs/290(GaCDP_CellTemp_C(26)) -> Input Conversion Subsystem/290(Inport_290)
  Harness Inputs/291(GaCDP_CellTemp_C(27)) -> Input Conversion Subsystem/291(Inport_291)
  Harness Inputs/292(GaCDP_CellTemp_C(28)) -> Input Conversion Subsystem/292(Inport_292)
  Harness Inputs/293(GaCDP_CellTemp_C(29)) -> Input Conversion Subsystem/293(Inport_293)
  Harness Inputs/294(GaCDP_CellTemp_C(30)) -> Input Conversion Subsystem/294(Inport_294)
  Harness Inputs/295(GaCDP_CellTemp_C(31)) -> Input Conversion Subsystem/295(Inport_295)
  Harness Inputs/296(GaCDP_CellTemp_C(32)) -> Input Conversion Subsystem/296(Inport_296)
  Harness Inputs/297(GaCDP_CellTemp_C(33)) -> Input Conversion Subsystem/297(Inport_297)
  Harness Inputs/298(GaCDP_CellTemp_C(34)) -> Input Conversion Subsystem/298(Inport_298)
  Harness Inputs/299(GaCDP_CellTemp_C(35)) -> Input Conversion Subsystem/299(Inport_299)
  Harness Inputs/300(GaCDP_CellTemp_C(36)) -> Input Conversion Subsystem/300(Inport_300)
  Harness Inputs/301(GaCDP_CellTemp_C(37)) -> Input Conversion Subsystem/301(Inport_301)
  Harness Inputs/302(GaCDP_CellTemp_C(38)) -> Input Conversion Subsystem/302(Inport_302)
  Harness Inputs/303(GaCDP_CellTemp_C(39)) -> Input Conversion Subsystem/303(Inport_303)
  Harness Inputs/304(GaCDP_CellTemp_C(40)) -> Input Conversion Subsystem/304(Inport_304)
  Harness Inputs/305(GaCDP_CellTemp_C(41)) -> Input Conversion Subsystem/305(Inport_305)
  Harness Inputs/306(GaCDP_CellTemp_C(42)) -> Input Conversion Subsystem/306(Inport_306)
  Harness Inputs/307(GaCDP_CellTemp_C(43)) -> Input Conversion Subsystem/307(Inport_307)
  Harness Inputs/308(GaCDP_CellTemp_C(44)) -> Input Conversion Subsystem/308(Inport_308)
  Harness Inputs/309(GaCDP_CellTemp_C(45)) -> Input Conversion Subsystem/309(Inport_309)
  Harness Inputs/310(GaCDP_CellTemp_C(46)) -> Input Conversion Subsystem/310(Inport_310)
  Harness Inputs/311(GaCDP_CellTemp_C(47)) -> Input Conversion Subsystem/311(Inport_311)
  Harness Inputs/312(GaCDP_CellTemp_C(48)) -> Input Conversion Subsystem/312(Inport_312)
  Harness Inputs/313(GcLDP_lntWtTemp_C) -> Input Conversion Subsystem/313(Inport_313)
  Harness Inputs/314(GcLDP_OutWtTemp_C) -> Input Conversion Subsystem/314(Inport_314)
  Harness Inputs/315(GcBTM_CoolPwrReq_W) -> Input Conversion Subsystem/315(Inport_315)
  Harness Inputs/316(GcBTM_HeatPwrReq_W) -> Input Conversion Subsystem/316(Inport_316)
  Harness Inputs/317(GeBTM_CoolReq_enum) -> Input Conversion Subsystem/317(Inport_317)
  Harness Inputs/318(GeBTM_HeatReq_enum) -> Input Conversion Subsystem/318(Inport_318)
  Harness Inputs/319(GbODP_V2XDischrgCmd_flg) -> Input Conversion Subsystem/319(Inport_319)
  Harness Inputs/320(GeMSM_BMUState_enum) -> Input Conversion Subsystem/320(Inport_320)
  Harness Inputs/321(GcHDP_FuseVolt_V) -> Input Conversion Subsystem/321(Inport_321)
  Harness Inputs/322(GbADP_DischgReq_flg) -> Input Conversion Subsystem/322(Inport_322)
  Harness Inputs/323(GcHDP_PosCtlVolt_V) -> Input Conversion Subsystem/323(Inport_323)
  Harness Inputs/324(GcCDP_MaxCellVoltNumb_numb) -> Input Conversion Subsystem/324(Inport_324)
  Harness Inputs/325(GcCDP_MinCellVoltNumb_numb) -> Input Conversion Subsystem/325(Inport_325)
  Harness Inputs/326(GcCDP_MaxCellTempNumb_numb) -> Input Conversion Subsystem/326(Inport_326)
  Harness Inputs/327(GcCDP_MinCellTempNumb_numb) -> Input Conversion Subsystem/327(Inport_327)
  Harness Inputs/328(GbWSM_DCWkUpPrs_flg) -> Input Conversion Subsystem/328(Inport_328)
  Harness Inputs/329(GbACC_PreThmObcChrgCmd_flg) -> Input Conversion Subsystem/329(Inport_329)
  Harness Inputs/330(GbACC_PreThmRqst_flg) -> Input Conversion Subsystem/330(Inport_330)
  Harness Inputs/331(GcACC_PreThmCrntRqst_A) -> Input Conversion Subsystem/331(Inport_331)
  Harness Inputs/332(GcACC_PreThmVoltRqst_V) -> Input Conversion Subsystem/332(Inport_332)
  Harness Inputs/333(GbACC_PreHeatPrmt_flg) -> Input Conversion Subsystem/333(Inport_333)
  Harness Inputs/334(GbFTC_PowerDown_flg) -> Input Conversion Subsystem/334(Inport_334)
  Harness Inputs/335(GcBTM_CoolTempReq_C) -> Input Conversion Subsystem/335(Inport_335)
  Harness Inputs/336(GcBTM_HeatTempReq_C) -> Input Conversion Subsystem/336(Inport_336)
  Harness Inputs/337(GcACC_ChrgingTiRem_min) -> Input Conversion Subsystem/337(Inport_337)
  Harness Inputs/338(GcDCC_ChrgingTiRem_min) -> Input Conversion Subsystem/338(Inport_338)
  Harness Inputs/339(GeVDP_PreThmEna_enum) -> Input Conversion Subsystem/339(Inport_339)
  Harness Inputs/340(GcSOP_DischrgPwr_kW) -> Input Conversion Subsystem/340(Inport_340)
  Harness Inputs/341(GcSOP_ChrgPwr_kW) -> Input Conversion Subsystem/341(Inport_341)
  Harness Inputs/342(GcCDP_MaxBusbarTemp_C) -> Input Conversion Subsystem/342(Inport_342)
  Harness Inputs/343(GcCDP_MinBusbarTemp_C) -> Input Conversion Subsystem/343(Inport_343)
  Harness Inputs/344(GeDCC_DCChrgState_enum) -> Input Conversion Subsystem/344(Inport_344)
  Harness Inputs/345(GeLDP_ChrgGunConnSt_enum) -> Input Conversion Subsystem/345(Inport_345)
  Harness Inputs/346(GbISP_TFThmRnwyfDet_flg) -> Input Conversion Subsystem/346(Inport_346)
  Harness Inputs/347(GaCDP_BusbarTemp_C(1)) -> Input Conversion Subsystem/347(Inport_347)
  Harness Inputs/348(GaCDP_BusbarTemp_C(2)) -> Input Conversion Subsystem/348(Inport_348)
  Harness Inputs/349(GaCDP_BusbarTemp_C(3)) -> Input Conversion Subsystem/349(Inport_349)
  Harness Inputs/350(GaCDP_BusbarTemp_C(4)) -> Input Conversion Subsystem/350(Inport_350)
  Harness Inputs/351(GaCDP_BusbarTemp_C(5)) -> Input Conversion Subsystem/351(Inport_351)
  Harness Inputs/352(GaCDP_BusbarTemp_C(6)) -> Input Conversion Subsystem/352(Inport_352)
  Harness Inputs/353(GaCDP_BusbarTemp_C(7)) -> Input Conversion Subsystem/353(Inport_353)
  Harness Inputs/354(GaCDP_BusbarTemp_C(8)) -> Input Conversion Subsystem/354(Inport_354)
  Harness Inputs/355(GaCDP_BusbarTemp_C(9)) -> Input Conversion Subsystem/355(Inport_355)
  Harness Inputs/356(GaCDP_BusbarTemp_C(10)) -> Input Conversion Subsystem/356(Inport_356)
  Harness Inputs/357(GaCDP_BusbarTemp_C(11)) -> Input Conversion Subsystem/357(Inport_357)
  Harness Inputs/358(GaCDP_BusbarTemp_C(12)) -> Input Conversion Subsystem/358(Inport_358)
  Harness Inputs/359(GaCDP_BusbarTemp_C(13)) -> Input Conversion Subsystem/359(Inport_359)
  Harness Inputs/360(GaCDP_BusbarTemp_C(14)) -> Input Conversion Subsystem/360(Inport_360)
  Harness Inputs/361(GaCDP_BusbarTemp_C(15)) -> Input Conversion Subsystem/361(Inport_361)
  Harness Inputs/362(GaCDP_BusbarTemp_C(16)) -> Input Conversion Subsystem/362(Inport_362)
  Harness Inputs/363(GaCDP_BusbarTemp_C(17)) -> Input Conversion Subsystem/363(Inport_363)
  Harness Inputs/364(GaCDP_BusbarTemp_C(18)) -> Input Conversion Subsystem/364(Inport_364)
  Harness Inputs/365(GaCDP_BusbarTemp_C(19)) -> Input Conversion Subsystem/365(Inport_365)
  Harness Inputs/366(GaCDP_BusbarTemp_C(20)) -> Input Conversion Subsystem/366(Inport_366)
  Harness Inputs/367(GaCDP_BusbarTemp_C(21)) -> Input Conversion Subsystem/367(Inport_367)
  Harness Inputs/368(GaCDP_BusbarTemp_C(22)) -> Input Conversion Subsystem/368(Inport_368)
  Harness Inputs/369(GaCDP_BusbarTemp_C(23)) -> Input Conversion Subsystem/369(Inport_369)
  Harness Inputs/370(GaCDP_BusbarTemp_C(24)) -> Input Conversion Subsystem/370(Inport_370)
  Harness Inputs/371(GaCDP_BusbarTemp_C(25)) -> Input Conversion Subsystem/371(Inport_371)
  Harness Inputs/372(GaCDP_BusbarTemp_C(26)) -> Input Conversion Subsystem/372(Inport_372)
  Harness Inputs/373(GaCDP_BusbarTemp_C(27)) -> Input Conversion Subsystem/373(Inport_373)
  Harness Inputs/374(GaCDP_BusbarTemp_C(28)) -> Input Conversion Subsystem/374(Inport_374)
  Harness Inputs/375(GaCDP_BusbarTemp_C(29)) -> Input Conversion Subsystem/375(Inport_375)
  Harness Inputs/376(GaCDP_BusbarTemp_C(30)) -> Input Conversion Subsystem/376(Inport_376)
  Harness Inputs/377(GaCDP_BusbarTemp_C(31)) -> Input Conversion Subsystem/377(Inport_377)
  Harness Inputs/378(GaCDP_BusbarTemp_C(32)) -> Input Conversion Subsystem/378(Inport_378)
  Harness Inputs/379(GaCDP_BusbarTemp_C(33)) -> Input Conversion Subsystem/379(Inport_379)
  Harness Inputs/380(GaCDP_BusbarTemp_C(34)) -> Input Conversion Subsystem/380(Inport_380)
  Harness Inputs/381(GaCDP_BusbarTemp_C(35)) -> Input Conversion Subsystem/381(Inport_381)
  Harness Inputs/382(GaCDP_BusbarTemp_C(36)) -> Input Conversion Subsystem/382(Inport_382)
  Harness Inputs/383(GaCDP_BusbarTemp_C(37)) -> Input Conversion Subsystem/383(Inport_383)
  Harness Inputs/384(GaCDP_BusbarTemp_C(38)) -> Input Conversion Subsystem/384(Inport_384)
  Harness Inputs/385(GaCDP_BusbarTemp_C(39)) -> Input Conversion Subsystem/385(Inport_385)
  Harness Inputs/386(GaCDP_BusbarTemp_C(40)) -> Input Conversion Subsystem/386(Inport_386)
  Harness Inputs/387(GaCDP_BusbarTemp_C(41)) -> Input Conversion Subsystem/387(Inport_387)
  Harness Inputs/388(GaCDP_BusbarTemp_C(42)) -> Input Conversion Subsystem/388(Inport_388)
  Harness Inputs/389(GaCDP_BusbarTemp_C(43)) -> Input Conversion Subsystem/389(Inport_389)
  Harness Inputs/390(GaCDP_BusbarTemp_C(44)) -> Input Conversion Subsystem/390(Inport_390)
  Harness Inputs/391(GaCDP_BusbarTemp_C(45)) -> Input Conversion Subsystem/391(Inport_391)
  Harness Inputs/392(GaCDP_BusbarTemp_C(46)) -> Input Conversion Subsystem/392(Inport_392)
  Harness Inputs/393(GaCDP_BusbarTemp_C(47)) -> Input Conversion Subsystem/393(Inport_393)
  Harness Inputs/394(GaCDP_BusbarTemp_C(48)) -> Input Conversion Subsystem/394(Inport_394)
  Harness Inputs/395(GcUDS_CellTempNumb_numb) -> Input Conversion Subsystem/395(Inport_395)
  Harness Inputs/396(GcUDS_BusbarTempNumb_numb) -> Input Conversion Subsystem/396(Inport_396)
  Harness Inputs/397(GcUDS_CellVoltNum_numb) -> Input Conversion Subsystem/397(Inport_397)
  Harness Inputs/398(GcUDS_BatEnergy_kWh) -> Input Conversion Subsystem/398(Inport_398)
  Harness Inputs/399(GbACC_HoldTempPrmt_flg) -> Input Conversion Subsystem/399(Inport_399)
  Harness Inputs/400(GbACC_HoldTempObcChrgCmd_flg) -> Input Conversion Subsystem/400(Inport_400)
  Harness Inputs/401(GcACC_HoldTempVoltRqst_V) -> Input Conversion Subsystem/401(Inport_401)
  Harness Inputs/402(GcACC_HoldTempCrntRqst_A) -> Input Conversion Subsystem/402(Inport_402)
  Harness Inputs/403(GbACC_HoldTempRqst_flg) -> Input Conversion Subsystem/403(Inport_403)
  Harness Inputs/404(GbISP_TFIsoResFltLevel2_flg) -> Input Conversion Subsystem/404(Inport_404)
  Harness Inputs/405(GbISP_TFIsoDCResFltLevel2_flg) -> Input Conversion Subsystem/405(Inport_405)
  Harness Inputs/406(GbISP_TFIsoHVoffResFltLevel2_flg) -> Input Conversion Subsystem/406(Inport_406)
  Harness Inputs/407(GbISP_TFIsoResFltLevel1_flg) -> Input Conversion Subsystem/407(Inport_407)
  Harness Inputs/408(GbISP_TFIsoDCResFltLevel1_flg) -> Input Conversion Subsystem/408(Inport_408)
  Harness Inputs/409(GbISP_TFIsoHVoffResFltLevel1_flg) -> Input Conversion Subsystem/409(Inport_409)
  Harness Inputs/410(GbADP_OTAmodeONReq_flg) -> Input Conversion Subsystem/410(Inport_410)
  Harness Inputs/411(GeUDS_AreaSel_enum) -> Input Conversion Subsystem/411(Inport_411)
  Harness Inputs/412(GeDCC_ElockReq_enum) -> Input Conversion Subsystem/412(Inport_412)
  Harness Inputs/413(GeTRA_ThmRnwySt_enum) -> Input Conversion Subsystem/413(Inport_413)
  Output Conversion Subsystem/1(Outport_1) -> GeCMS_HVConnSt_enum/1
  Output Conversion Subsystem/2(Outport_2) -> GbCMS_NegCtlSt_flg/1
  Output Conversion Subsystem/3(Outport_3) -> GbCMS_PosCtlSt_flg/1
  Output Conversion Subsystem/4(Outport_4) -> GbCMS_ChrgPosCtlSt_flg/1
  Output Conversion Subsystem/5(Outport_5) -> GbCMS_ChrgNegCtlSt_flg/1
  Output Conversion Subsystem/6(Outport_6) -> GeCMS_RelStuckClosed_enum/1
  Output Conversion Subsystem/7(Outport_7) -> GcCMS_PackVolt_V/1
  Output Conversion Subsystem/8(Outport_8) -> GbCMS_PreChrgCtlSt_flg/1
  Output Conversion Subsystem/9(Outport_9) -> GcCMS_BattCurr_A/1
  Output Conversion Subsystem/10(Outport_10) -> GbCMS_Kl15WkUp_flg/1
  Output Conversion Subsystem/11(Outport_11) -> GbCMS_ThmRunAway_flg/1
  Output Conversion Subsystem/12(Outport_12) -> GcCMS_CoolTempIn_C/1
  Output Conversion Subsystem/13(Outport_13) -> GcCMS_CoolTempOut_C/1
  Output Conversion Subsystem/14(Outport_14) -> GcCMS_CoolPwrReq_W/1
  Output Conversion Subsystem/15(Outport_15) -> GcCMS_HeatPwrReq_W/1
  Output Conversion Subsystem/16(Outport_16) -> GeCMS_CoolReq_enum/1
  Output Conversion Subsystem/17(Outport_17) -> GeCMS_HeatReq_enum/1
  Output Conversion Subsystem/18(Outport_18) -> GcCMS_PeakCurrDisCh_A/1
  Output Conversion Subsystem/19(Outport_19) -> GcCMS_PeakCurrCh_A/1
  Output Conversion Subsystem/20(Outport_20) -> GcCMS_PeakVoltDisCh_V/1
  Output Conversion Subsystem/21(Outport_21) -> GcCMS_PeakVoltCh_V/1
  Output Conversion Subsystem/22(Outport_22) -> GeCMS_Thm_propagat_enum/1
  Output Conversion Subsystem/23(Outport_23) -> GcCMS_ClntTgtTemp_C/1
  Output Conversion Subsystem/24(Outport_24) -> GcCMS_HtTgtTemp_C/1
  Output Conversion Subsystem/25(Outport_25) -> GcCMS_MaxCellVolt_V/1
  Output Conversion Subsystem/26(Outport_26) -> GcCMS_BusbarTempMax_C/1
  Output Conversion Subsystem/27(Outport_27) -> GcCMS_BusbarTempMin_C/1
  Output Conversion Subsystem/28(Outport_28) -> GcCMS_MinCellVolt_V/1
  Output Conversion Subsystem/29(Outport_29) -> GbCMS_ChrgCmd_flg/1
  Output Conversion Subsystem/30(Outport_30) -> GcCMS_ActPwrChrg_Kw/1
  Output Conversion Subsystem/31(Outport_31) -> GcCMS_MaxVoltChrg_V/1
  Output Conversion Subsystem/32(Outport_32) -> GcCMS_ReqVoltChrg_V/1
  Output Conversion Subsystem/33(Outport_33) -> GcCMS_ReqCurrChrg_A/1
  Output Conversion Subsystem/34(Outport_34) -> GbCMS_ObcRdyReq_flg/1
  Output Conversion Subsystem/35(Outport_35) -> GbCMS_DischgCmd_flg/1
  Output Conversion Subsystem/36(Outport_36) -> GeCMS_BmsSt_enum/1
  Output Conversion Subsystem/37(Outport_37) -> GeCMS_BmsSelfChk_enum/1
  Output Conversion Subsystem/38(Outport_38) -> GeCMS_IsoFault_enum/1
  Output Conversion Subsystem/39(Outport_39) -> GcCMS_SocDspl_pct/1
  Output Conversion Subsystem/40(Outport_40) -> GbCMS_HvilOpenFault_flg/1
  Output Conversion Subsystem/41(Outport_41) -> GeCMS_FltLvl_enum/1
  Output Conversion Subsystem/42(Outport_42) -> GeCMS_V2xMod_enum/1
  Output Conversion Subsystem/43(Outport_43) -> GcCMS_ChgSOCset_pct/1
  Output Conversion Subsystem/44(Outport_44) -> GcCMS_BattSoh_pct/1
  Output Conversion Subsystem/45(Outport_45) -> GcCMS_SOCA_pct/1
  Output Conversion Subsystem/46(Outport_46) -> GeCMS_IviDischg_enum/1
  Output Conversion Subsystem/47(Outport_47) -> GcCMS_PackCurLem_A/1
  Output Conversion Subsystem/48(Outport_48) -> GcCMS_BattInVolt_V/1
  Output Conversion Subsystem/49(Outport_49) -> GbCMS_BalSt_flg/1
  Output Conversion Subsystem/50(Outport_50) -> GbCMS_BalVlg_flg/1
  Output Conversion Subsystem/51(Outport_51) -> GbCMS_VcuPwrUpReq_flg/1
  Output Conversion Subsystem/52(Outport_52) -> GbCMS_VcuPwrUpReqVld_flg/1
  Output Conversion Subsystem/53(Outport_53) -> GcCMS_ConstCurrDisChMax_A/1
  Output Conversion Subsystem/54(Outport_54) -> GcCMS_ConstCurrChMax_A/1
  Output Conversion Subsystem/55(Outport_55) -> GbCMS_PwrDownReq_flg/1
  Output Conversion Subsystem/56(Outport_56) -> GbCMS_PwrDownReqVld_flg/1
  Output Conversion Subsystem/57(Outport_57) -> GeCMS_ChrgPreThmMode_enum/1
  Output Conversion Subsystem/58(Outport_58) -> GeCMS_ElockReq_enum/1
  Output Conversion Subsystem/59(Outport_59) -> GeCMS_PreThmReq_enum/1
  Output Conversion Subsystem/60(Outport_60) -> GcCMS_PeakPwrDisCh_Kw/1
  Output Conversion Subsystem/61(Outport_61) -> GcCMS_PeakPwrCh_Kw/1
  Output Conversion Subsystem/62(Outport_62) -> GcCMS_ConstPwrDisCh_Kw/1
  Output Conversion Subsystem/63(Outport_63) -> GcCMS_ConstPwrCh_Kw/1
  Output Conversion Subsystem/64(Outport_64) -> GcCMS_ResIso_Kohm/1
  Output Conversion Subsystem/65(Outport_65) -> GcCMS_ChrgRemTime_Min/1
  Output Conversion Subsystem/66(Outport_66) -> GeCMS_ACPlugCnnt_enum/1
  Output Conversion Subsystem/67(Outport_67) -> GbCMS_BattFull_flg/1
  Output Conversion Subsystem/68(Outport_68) -> GbCMS_WarnLamp_flg/1
  Output Conversion Subsystem/69(Outport_69) -> GbCMS_SerLamp_flg/1
  Output Conversion Subsystem/70(Outport_70) -> GbCMS_TempDiffWarn_flg/1
  Output Conversion Subsystem/71(Outport_71) -> GbCMS_OverChrgWarn_flg/1
  Output Conversion Subsystem/72(Outport_72) -> GbCMS_ConsisWarn_flg/1
  Output Conversion Subsystem/73(Outport_73) -> GbCMS_MishWarn_flg/1
  Output Conversion Subsystem/74(Outport_74) -> GbCMS_SocHopWarn_flg/1
  Output Conversion Subsystem/75(Outport_75) -> GbCMS_SocHighWarn_flg/1
  Output Conversion Subsystem/76(Outport_76) -> GbCMS_SocLowWarn_flg/1
  Output Conversion Subsystem/77(Outport_77) -> GbCMS_OTAModeSt_flg/1
  Output Conversion Subsystem/78(Outport_78) -> GeCMS_AcDcConnBoth_enum/1
  Output Conversion Subsystem/79(Outport_79) -> GbCMS_CellUvFlt_flg/1
  Output Conversion Subsystem/80(Outport_80) -> GbCMS_CellOvFlt_flg/1
  Output Conversion Subsystem/81(Outport_81) -> GbCMS_PackUvFlt_flg/1
  Output Conversion Subsystem/82(Outport_82) -> GbCMS_PackOvFlt_flg/1
  Output Conversion Subsystem/83(Outport_83) -> GbCMS_TempHighWarn_flg/1
  Output Conversion Subsystem/84(Outport_84) -> GcCMS_RealSoc_pct/1
  Output Conversion Subsystem/85(Outport_85) -> GeCMS_DCPlugConn_enum/1
  Output Conversion Subsystem/86(Outport_86) -> GeCMS_ACChgMode_enum/1
  Output Conversion Subsystem/87(Outport_87) -> GeCMS_DCChgMode_enum/1
  Output Conversion Subsystem/88(Outport_88) -> GcCMS_BattTempAvrg_C/1
  Output Conversion Subsystem/89(Outport_89) -> GcCMS_BattNrmEnrg_kwh/1
  Output Conversion Subsystem/90(Outport_90) -> GbCMS_BattTempFault_flg/1
  Output Conversion Subsystem/91(Outport_91) -> GcCMS_BattSoe_kwh/1
  Output Conversion Subsystem/92(Outport_92) -> GbCMS_IsoChkSt_flg/1
  Output Conversion Subsystem/93(Outport_93) -> GcCMS_BattTempMax_C/1
  Output Conversion Subsystem/94(Outport_94) -> GcCMS_BattTempMin_C/1
  Output Conversion Subsystem/95(Outport_95) -> GcCMS_FuseVolt_V/1
  Output Conversion Subsystem/96(Outport_96) -> GcCMS_ChrgAccum_Ah/1
  Output Conversion Subsystem/97(Outport_97) -> GbCMS_DChgStVoltOut_flg/1
  Output Conversion Subsystem/98(Outport_98) -> GcCMS_DChrgVoltReq_V/1
  Output Conversion Subsystem/99(Outport_99) -> GcCMS_DChrgCurrReq_A/1
  Output Conversion Subsystem/100(Outport_100) -> GcCMS_DChrgRchSocLmt_numb/1
  Output Conversion Subsystem/101(Outport_101) -> GcCMS_DChrgRchPackVoltLmt_numb/1
  Output Conversion Subsystem/102(Outport_102) -> GcCMS_DChrgRchCellVoltLmt_numb/1
  Output Conversion Subsystem/103(Outport_103) -> GcCMS_DChrgChrgerActStop_numb/1
  Output Conversion Subsystem/104(Outport_104) -> GcCMS_DChrgBattInsulationErr_numb/1
  Output Conversion Subsystem/105(Outport_105) -> GcCMS_DChrgOutpCnntOvrTempErr_numb/1
  Output Conversion Subsystem/106(Outport_106) -> GcCMS_PcbOvrTempErr_numb/1
  Output Conversion Subsystem/107(Outport_107) -> GcCMS_ChrgCnntErr_numb/1
  Output Conversion Subsystem/108(Outport_108) -> GcCMS_BattOvrTempErr_numb/1
  Output Conversion Subsystem/109(Outport_109) -> GcCMS_MainRelayErr_numb/1
  Output Conversion Subsystem/110(Outport_110) -> GcCMS_CC2ChkVoltErr_numb/1
  Output Conversion Subsystem/111(Outport_111) -> GcCMS_OtherErr_numb/1
  Output Conversion Subsystem/112(Outport_112) -> GcCMS_ChrgCurrAbnrm_numb/1
  Output Conversion Subsystem/113(Outport_113) -> GcCMS_ChrgVoltAbnrm_numb/1
  Output Conversion Subsystem/114(Outport_114) -> GcCMS_CellVoltCnt_numb/1
  Output Conversion Subsystem/115(Outport_115) -> GcCMS_CellVolt1_V/1
  Output Conversion Subsystem/116(Outport_116) -> GcCMS_CellVolt2_V/1
  Output Conversion Subsystem/117(Outport_117) -> GcCMS_CellVolt3_V/1
  Output Conversion Subsystem/118(Outport_118) -> GcCMS_CellVolt4_V/1
  Output Conversion Subsystem/119(Outport_119) -> GcCMS_CellTempCnt_numb/1
  Output Conversion Subsystem/120(Outport_120) -> GcCMS_CellTemp1_C/1
  Output Conversion Subsystem/121(Outport_121) -> GcCMS_CellTemp2_C/1
  Output Conversion Subsystem/122(Outport_122) -> GcCMS_CellTemp3_C/1
  Output Conversion Subsystem/123(Outport_123) -> GcCMS_CellTemp4_C/1
  Output Conversion Subsystem/124(Outport_124) -> GcCMS_CellTemp5_C/1
  Output Conversion Subsystem/125(Outport_125) -> GcCMS_CellTemp6_C/1
  Output Conversion Subsystem/126(Outport_126) -> GcCMS_CellTemp7_C/1
  Output Conversion Subsystem/127(Outport_127) -> GcCMS_MaxCellVoltNumb_numb/1
  Output Conversion Subsystem/128(Outport_128) -> GcCMS_MinCellVoltNumb_numb/1
  Output Conversion Subsystem/129(Outport_129) -> GcCMS_MaxCellTempNumb_numb/1
  Output Conversion Subsystem/130(Outport_130) -> GcCMS_MinCellTempNumb_numb/1
  Output Conversion Subsystem/131(Outport_131) -> GcCMS_MaxVoltNumb_numb/1
  Output Conversion Subsystem/132(Outport_132) -> GcCMS_MinVoltNumb_numb/1
  Output Conversion Subsystem/133(Outport_133) -> GcCMS_MaxTempNumb_numb/1
  Output Conversion Subsystem/134(Outport_134) -> GcCMS_MinTempNumb_numb/1
  Output Conversion Subsystem/135(Outport_135) -> GeCMS_ChgMode_enum/1
  Output Conversion Subsystem/136(Outport_136) -> GeCMS_DChrgModeDebug_enum/1
  Output Conversion Subsystem/137(Outport_137) -> GbCMS_DChrgWkUp_flg/1
  Output Conversion Subsystem/138(Outport_138) -> GeCMS_EvccMode_enum/1
  Output Conversion Subsystem/139(Outport_139) -> GeCMS_AChrgObsr_enum/1
  Output Conversion Subsystem/140(Outport_140) -> GeCMS_PreThmObsvr_enum/1
  Output Conversion Subsystem/141(Outport_141) -> GbCMS_StartCanSend_flg/1
  Output Conversion Subsystem/142(Outport_142) -> GeCMS_AppChgMode_enum/1
  Output Conversion Subsystem/143(Outport_143) -> GeCMS_DCchgIsolationFault_enum/1
  Input Conversion Subsystem/1(Outport_1) -> CMS_MIL/1
  Input Conversion Subsystem/2(Outport_2) -> CMS_MIL/2
  Input Conversion Subsystem/3(Outport_3) -> CMS_MIL/3
  Input Conversion Subsystem/4(Outport_4) -> CMS_MIL/4
  Input Conversion Subsystem/5(Outport_5) -> CMS_MIL/5
  Input Conversion Subsystem/6(Outport_6) -> CMS_MIL/6
  Input Conversion Subsystem/7(Outport_7) -> CMS_MIL/7
  Input Conversion Subsystem/8(Outport_8) -> CMS_MIL/8
  Input Conversion Subsystem/9(Outport_9) -> CMS_MIL/9
  Input Conversion Subsystem/10(Outport_10) -> CMS_MIL/10
  Input Conversion Subsystem/11(Outport_11) -> CMS_MIL/11
  Input Conversion Subsystem/12(Outport_12) -> CMS_MIL/12
  Input Conversion Subsystem/13(Outport_13) -> CMS_MIL/13
  Input Conversion Subsystem/14(Outport_14) -> CMS_MIL/14
  Input Conversion Subsystem/15(Outport_15) -> CMS_MIL/15
  Input Conversion Subsystem/16(Outport_16) -> CMS_MIL/16
  Input Conversion Subsystem/17(Outport_17) -> CMS_MIL/17
  Input Conversion Subsystem/18(Outport_18) -> CMS_MIL/18
  Input Conversion Subsystem/19(Outport_19) -> CMS_MIL/19
  Input Conversion Subsystem/20(Outport_20) -> CMS_MIL/20
  Input Conversion Subsystem/21(Outport_21) -> CMS_MIL/21
  Input Conversion Subsystem/22(Outport_22) -> CMS_MIL/22
  Input Conversion Subsystem/23(Outport_23) -> CMS_MIL/23
  Input Conversion Subsystem/24(Outport_24) -> CMS_MIL/24
  Input Conversion Subsystem/25(Outport_25) -> CMS_MIL/25
  Input Conversion Subsystem/26(Outport_26) -> CMS_MIL/26
  Input Conversion Subsystem/27(Outport_27) -> CMS_MIL/27
  Input Conversion Subsystem/28(Outport_28) -> CMS_MIL/28
  Input Conversion Subsystem/29(Outport_29) -> CMS_MIL/29
  Input Conversion Subsystem/30(Outport_30) -> CMS_MIL/30
  Input Conversion Subsystem/31(Outport_31) -> CMS_MIL/31
  Input Conversion Subsystem/32(Outport_32) -> CMS_MIL/32
  Input Conversion Subsystem/33(Outport_33) -> CMS_MIL/33
  Input Conversion Subsystem/34(Outport_34) -> CMS_MIL/34
  Input Conversion Subsystem/35(Outport_35) -> CMS_MIL/35
  Input Conversion Subsystem/36(Outport_36) -> CMS_MIL/36
  Input Conversion Subsystem/37(Outport_37) -> CMS_MIL/37
  Input Conversion Subsystem/38(Outport_38) -> CMS_MIL/38
  Input Conversion Subsystem/39(Outport_39) -> CMS_MIL/39
  Input Conversion Subsystem/40(Outport_40) -> CMS_MIL/40
  Input Conversion Subsystem/41(Outport_41) -> CMS_MIL/41
  Input Conversion Subsystem/42(Outport_42) -> CMS_MIL/42
  Input Conversion Subsystem/43(Outport_43) -> CMS_MIL/43
  Input Conversion Subsystem/44(Outport_44) -> CMS_MIL/44
  Input Conversion Subsystem/45(Outport_45) -> CMS_MIL/45
  Input Conversion Subsystem/46(Outport_46) -> CMS_MIL/46
  Input Conversion Subsystem/47(Outport_47) -> CMS_MIL/47
  Input Conversion Subsystem/48(Outport_48) -> CMS_MIL/48
  Input Conversion Subsystem/49(Outport_49) -> CMS_MIL/49
  Input Conversion Subsystem/50(Outport_50) -> CMS_MIL/50
  Input Conversion Subsystem/51(Outport_51) -> CMS_MIL/51
  Input Conversion Subsystem/52(Outport_52) -> CMS_MIL/52
  Input Conversion Subsystem/53(Outport_53) -> CMS_MIL/53
  Input Conversion Subsystem/54(Outport_54) -> CMS_MIL/54
  Input Conversion Subsystem/55(Outport_55) -> CMS_MIL/55
  Input Conversion Subsystem/56(Outport_56) -> CMS_MIL/56
  Input Conversion Subsystem/57(Outport_57) -> CMS_MIL/57
  Input Conversion Subsystem/58(Outport_58) -> CMS_MIL/58
  Input Conversion Subsystem/59(Outport_59) -> CMS_MIL/59
  Input Conversion Subsystem/60(Outport_60) -> CMS_MIL/60
  Input Conversion Subsystem/61(Outport_61) -> CMS_MIL/61
  Input Conversion Subsystem/62(Outport_62) -> CMS_MIL/62
  Input Conversion Subsystem/63(Outport_63) -> CMS_MIL/63
  Input Conversion Subsystem/64(Outport_64) -> CMS_MIL/64
  Input Conversion Subsystem/65(Outport_65) -> CMS_MIL/65
  Input Conversion Subsystem/66(Outport_66) -> CMS_MIL/66
  Input Conversion Subsystem/67(Outport_67) -> CMS_MIL/67
  Input Conversion Subsystem/68(Outport_68) -> CMS_MIL/68
  Input Conversion Subsystem/69(Outport_69) -> CMS_MIL/69
  Input Conversion Subsystem/70(Outport_70) -> CMS_MIL/70
  Input Conversion Subsystem/71(Outport_71) -> CMS_MIL/71
  Input Conversion Subsystem/72(Outport_72) -> CMS_MIL/72
  Input Conversion Subsystem/73(Outport_73) -> CMS_MIL/73
  Input Conversion Subsystem/74(Outport_74) -> CMS_MIL/74
  Input Conversion Subsystem/75(Outport_75) -> CMS_MIL/75
  Input Conversion Subsystem/76(Outport_76) -> CMS_MIL/76
  Input Conversion Subsystem/77(Outport_77) -> CMS_MIL/77
  Input Conversion Subsystem/78(Outport_78) -> CMS_MIL/78
  Input Conversion Subsystem/79(Outport_79) -> CMS_MIL/79
  Input Conversion Subsystem/80(Outport_80) -> CMS_MIL/80
  Input Conversion Subsystem/81(Outport_81) -> CMS_MIL/81
  Input Conversion Subsystem/82(Outport_82) -> CMS_MIL/82
  Input Conversion Subsystem/83(Outport_83) -> CMS_MIL/83
  Input Conversion Subsystem/84(Outport_84) -> CMS_MIL/84
  Input Conversion Subsystem/85(Outport_85) -> CMS_MIL/85
  Input Conversion Subsystem/86(Outport_86) -> CMS_MIL/86
  Input Conversion Subsystem/87(Outport_87) -> CMS_MIL/87
  Input Conversion Subsystem/88(Outport_88) -> CMS_MIL/88
  Input Conversion Subsystem/89(Outport_89) -> CMS_MIL/89
  Input Conversion Subsystem/90(Outport_90) -> CMS_MIL/90
  Input Conversion Subsystem/91(Outport_91) -> CMS_MIL/91
  Input Conversion Subsystem/92(Outport_92) -> CMS_MIL/92
  Input Conversion Subsystem/93(Outport_93) -> CMS_MIL/93
  Input Conversion Subsystem/94(Outport_94) -> CMS_MIL/94
  Input Conversion Subsystem/95(Outport_95) -> CMS_MIL/95
  Input Conversion Subsystem/96(Outport_96) -> CMS_MIL/96
  Input Conversion Subsystem/97(Outport_97) -> CMS_MIL/97
  CMS_MIL/1 -> Output Conversion Subsystem/1(Inport_1)
  CMS_MIL/2 -> Output Conversion Subsystem/2(Inport_2)
  CMS_MIL/3 -> Output Conversion Subsystem/3(Inport_3)
  CMS_MIL/4 -> Output Conversion Subsystem/4(Inport_4)
  CMS_MIL/5 -> Output Conversion Subsystem/5(Inport_5)
  CMS_MIL/6 -> Output Conversion Subsystem/6(Inport_6)
  CMS_MIL/7 -> Output Conversion Subsystem/7(Inport_7)
  CMS_MIL/8 -> Output Conversion Subsystem/8(Inport_8)
  CMS_MIL/9 -> Output Conversion Subsystem/9(Inport_9)
  CMS_MIL/10 -> Output Conversion Subsystem/10(Inport_10)
  CMS_MIL/11 -> Output Conversion Subsystem/11(Inport_11)
  CMS_MIL/12 -> Output Conversion Subsystem/12(Inport_12)
  CMS_MIL/13 -> Output Conversion Subsystem/13(Inport_13)
  CMS_MIL/14 -> Output Conversion Subsystem/14(Inport_14)
  CMS_MIL/15 -> Output Conversion Subsystem/15(Inport_15)
  CMS_MIL/16 -> Output Conversion Subsystem/16(Inport_16)
  CMS_MIL/17 -> Output Conversion Subsystem/17(Inport_17)
  CMS_MIL/18 -> Output Conversion Subsystem/18(Inport_18)
  CMS_MIL/19 -> Output Conversion Subsystem/19(Inport_19)
  CMS_MIL/20 -> Output Conversion Subsystem/20(Inport_20)
  CMS_MIL/21 -> Output Conversion Subsystem/21(Inport_21)
  CMS_MIL/22 -> Output Conversion Subsystem/22(Inport_22)
  CMS_MIL/23 -> Output Conversion Subsystem/23(Inport_23)
  CMS_MIL/24 -> Output Conversion Subsystem/24(Inport_24)
  CMS_MIL/25 -> Output Conversion Subsystem/25(Inport_25)
  CMS_MIL/26 -> Output Conversion Subsystem/26(Inport_26)
  CMS_MIL/27 -> Output Conversion Subsystem/27(Inport_27)
  CMS_MIL/28 -> Output Conversion Subsystem/28(Inport_28)
  CMS_MIL/29 -> Output Conversion Subsystem/29(Inport_29)
  CMS_MIL/30 -> Output Conversion Subsystem/30(Inport_30)
  CMS_MIL/31 -> Output Conversion Subsystem/31(Inport_31)
  CMS_MIL/32 -> Output Conversion Subsystem/32(Inport_32)
  CMS_MIL/33 -> Output Conversion Subsystem/33(Inport_33)
  CMS_MIL/34 -> Output Conversion Subsystem/34(Inport_34)
  CMS_MIL/35 -> Output Conversion Subsystem/35(Inport_35)
  CMS_MIL/36 -> Output Conversion Subsystem/36(Inport_36)
  CMS_MIL/37 -> Output Conversion Subsystem/37(Inport_37)
  CMS_MIL/38 -> Output Conversion Subsystem/38(Inport_38)
  CMS_MIL/39 -> Output Conversion Subsystem/39(Inport_39)
  CMS_MIL/40 -> Output Conversion Subsystem/40(Inport_40)
  CMS_MIL/41 -> Output Conversion Subsystem/41(Inport_41)
  CMS_MIL/42 -> Output Conversion Subsystem/42(Inport_42)
  CMS_MIL/43 -> Output Conversion Subsystem/43(Inport_43)
  CMS_MIL/44 -> Output Conversion Subsystem/44(Inport_44)
  CMS_MIL/45 -> Output Conversion Subsystem/45(Inport_45)
  CMS_MIL/46 -> Output Conversion Subsystem/46(Inport_46)
  CMS_MIL/47 -> Output Conversion Subsystem/47(Inport_47)
  CMS_MIL/48 -> Output Conversion Subsystem/48(Inport_48)
  CMS_MIL/49 -> Output Conversion Subsystem/49(Inport_49)
  CMS_MIL/50 -> Output Conversion Subsystem/50(Inport_50)
  CMS_MIL/51 -> Output Conversion Subsystem/51(Inport_51)
  CMS_MIL/52 -> Output Conversion Subsystem/52(Inport_52)
  CMS_MIL/53 -> Output Conversion Subsystem/53(Inport_53)
  CMS_MIL/54 -> Output Conversion Subsystem/54(Inport_54)
  CMS_MIL/55 -> Output Conversion Subsystem/55(Inport_55)
  CMS_MIL/56 -> Output Conversion Subsystem/56(Inport_56)
  CMS_MIL/57 -> Output Conversion Subsystem/57(Inport_57)
  CMS_MIL/58 -> Output Conversion Subsystem/58(Inport_58)
  CMS_MIL/59 -> Output Conversion Subsystem/59(Inport_59)
  CMS_MIL/60 -> Output Conversion Subsystem/60(Inport_60)
  CMS_MIL/61 -> Output Conversion Subsystem/61(Inport_61)
  CMS_MIL/62 -> Output Conversion Subsystem/62(Inport_62)
  CMS_MIL/63 -> Output Conversion Subsystem/63(Inport_63)
  CMS_MIL/64 -> Output Conversion Subsystem/64(Inport_64)
  CMS_MIL/65 -> Output Conversion Subsystem/65(Inport_65)
  CMS_MIL/66 -> Output Conversion Subsystem/66(Inport_66)
  CMS_MIL/67 -> Output Conversion Subsystem/67(Inport_67)
  CMS_MIL/68 -> Output Conversion Subsystem/68(Inport_68)
  CMS_MIL/69 -> Output Conversion Subsystem/69(Inport_69)
  CMS_MIL/70 -> Output Conversion Subsystem/70(Inport_70)
  CMS_MIL/71 -> Output Conversion Subsystem/71(Inport_71)
  CMS_MIL/72 -> Output Conversion Subsystem/72(Inport_72)
  CMS_MIL/73 -> Output Conversion Subsystem/73(Inport_73)
  CMS_MIL/74 -> Output Conversion Subsystem/74(Inport_74)
  CMS_MIL/75 -> Output Conversion Subsystem/75(Inport_75)
  CMS_MIL/76 -> Output Conversion Subsystem/76(Inport_76)
  CMS_MIL/77 -> Output Conversion Subsystem/77(Inport_77)
  CMS_MIL/78 -> Output Conversion Subsystem/78(Inport_78)
  CMS_MIL/79 -> Output Conversion Subsystem/79(Inport_79)
  CMS_MIL/80 -> Output Conversion Subsystem/80(Inport_80)
  CMS_MIL/81 -> Output Conversion Subsystem/81(Inport_81)
  CMS_MIL/82 -> Output Conversion Subsystem/82(Inport_82)
  CMS_MIL/83 -> Output Conversion Subsystem/83(Inport_83)
  CMS_MIL/84 -> Output Conversion Subsystem/84(Inport_84)
  CMS_MIL/85 -> Output Conversion Subsystem/85(Inport_85)
  CMS_MIL/86 -> Output Conversion Subsystem/86(Inport_86)
  CMS_MIL/87 -> Output Conversion Subsystem/87(Inport_87)
  CMS_MIL/88 -> Output Conversion Subsystem/88(Inport_88)
  CMS_MIL/89 -> Output Conversion Subsystem/89(Inport_89)
  CMS_MIL/90 -> Output Conversion Subsystem/90(Inport_90)
  CMS_MIL/91 -> Output Conversion Subsystem/91(Inport_91)
  CMS_MIL/92 -> Output Conversion Subsystem/92(Inport_92)
  CMS_MIL/93 -> Output Conversion Subsystem/93(Inport_93)
  CMS_MIL/94 -> Output Conversion Subsystem/94(Inport_94)
  CMS_MIL/95 -> Output Conversion Subsystem/95(Inport_95)
  CMS_MIL/96 -> Output Conversion Subsystem/96(Inport_96)
  CMS_MIL/97 -> Output Conversion Subsystem/97(Inport_97)
  CMS_MIL/98 -> Output Conversion Subsystem/98(Inport_98)
  CMS_MIL/99 -> Output Conversion Subsystem/99(Inport_99)
  CMS_MIL/100 -> Output Conversion Subsystem/100(Inport_100)
  CMS_MIL/101 -> Output Conversion Subsystem/101(Inport_101)
  CMS_MIL/102 -> Output Conversion Subsystem/102(Inport_102)
  CMS_MIL/103 -> Output Conversion Subsystem/103(Inport_103)
  CMS_MIL/104 -> Output Conversion Subsystem/104(Inport_104)
  CMS_MIL/105 -> Output Conversion Subsystem/105(Inport_105)
  CMS_MIL/106 -> Output Conversion Subsystem/106(Inport_106)
  CMS_MIL/107 -> Output Conversion Subsystem/107(Inport_107)
  CMS_MIL/108 -> Output Conversion Subsystem/108(Inport_108)
  CMS_MIL/109 -> Output Conversion Subsystem/109(Inport_109)
  CMS_MIL/110 -> Output Conversion Subsystem/110(Inport_110)
  CMS_MIL/111 -> Output Conversion Subsystem/111(Inport_111)
  CMS_MIL/112 -> Output Conversion Subsystem/112(Inport_112)
  CMS_MIL/113 -> Output Conversion Subsystem/113(Inport_113)
  CMS_MIL/114 -> Output Conversion Subsystem/114(Inport_114)
  CMS_MIL/115 -> Output Conversion Subsystem/115(Inport_115)
  CMS_MIL/116 -> Output Conversion Subsystem/116(Inport_116)
  CMS_MIL/117 -> Output Conversion Subsystem/117(Inport_117)
  CMS_MIL/118 -> Output Conversion Subsystem/118(Inport_118)
  CMS_MIL/119 -> Output Conversion Subsystem/119(Inport_119)
  CMS_MIL/120 -> Output Conversion Subsystem/120(Inport_120)
  CMS_MIL/121 -> Output Conversion Subsystem/121(Inport_121)
  CMS_MIL/122 -> Output Conversion Subsystem/122(Inport_122)
  CMS_MIL/123 -> Output Conversion Subsystem/123(Inport_123)
  CMS_MIL/124 -> Output Conversion Subsystem/124(Inport_124)
  CMS_MIL/125 -> Output Conversion Subsystem/125(Inport_125)
  CMS_MIL/126 -> Output Conversion Subsystem/126(Inport_126)
  CMS_MIL/127 -> Output Conversion Subsystem/127(Inport_127)
  CMS_MIL/128 -> Output Conversion Subsystem/128(Inport_128)
  CMS_MIL/129 -> Output Conversion Subsystem/129(Inport_129)
  CMS_MIL/130 -> Output Conversion Subsystem/130(Inport_130)
  CMS_MIL/131 -> Output Conversion Subsystem/131(Inport_131)
  CMS_MIL/132 -> Output Conversion Subsystem/132(Inport_132)
  CMS_MIL/133 -> Output Conversion Subsystem/133(Inport_133)
  CMS_MIL/134 -> Output Conversion Subsystem/134(Inport_134)
  CMS_MIL/135 -> Output Conversion Subsystem/135(Inport_135)
  CMS_MIL/136 -> Output Conversion Subsystem/136(Inport_136)
  CMS_MIL/137 -> Output Conversion Subsystem/137(Inport_137)
  CMS_MIL/138 -> Output Conversion Subsystem/138(Inport_138)
  CMS_MIL/139 -> Output Conversion Subsystem/139(Inport_139)
  CMS_MIL/140 -> Output Conversion Subsystem/140(Inport_140)
  CMS_MIL/141 -> Output Conversion Subsystem/141(Inport_141)
  CMS_MIL/142 -> Output Conversion Subsystem/142(Inport_142)
  CMS_MIL/143 -> Output Conversion Subsystem/143(Inport_143)
